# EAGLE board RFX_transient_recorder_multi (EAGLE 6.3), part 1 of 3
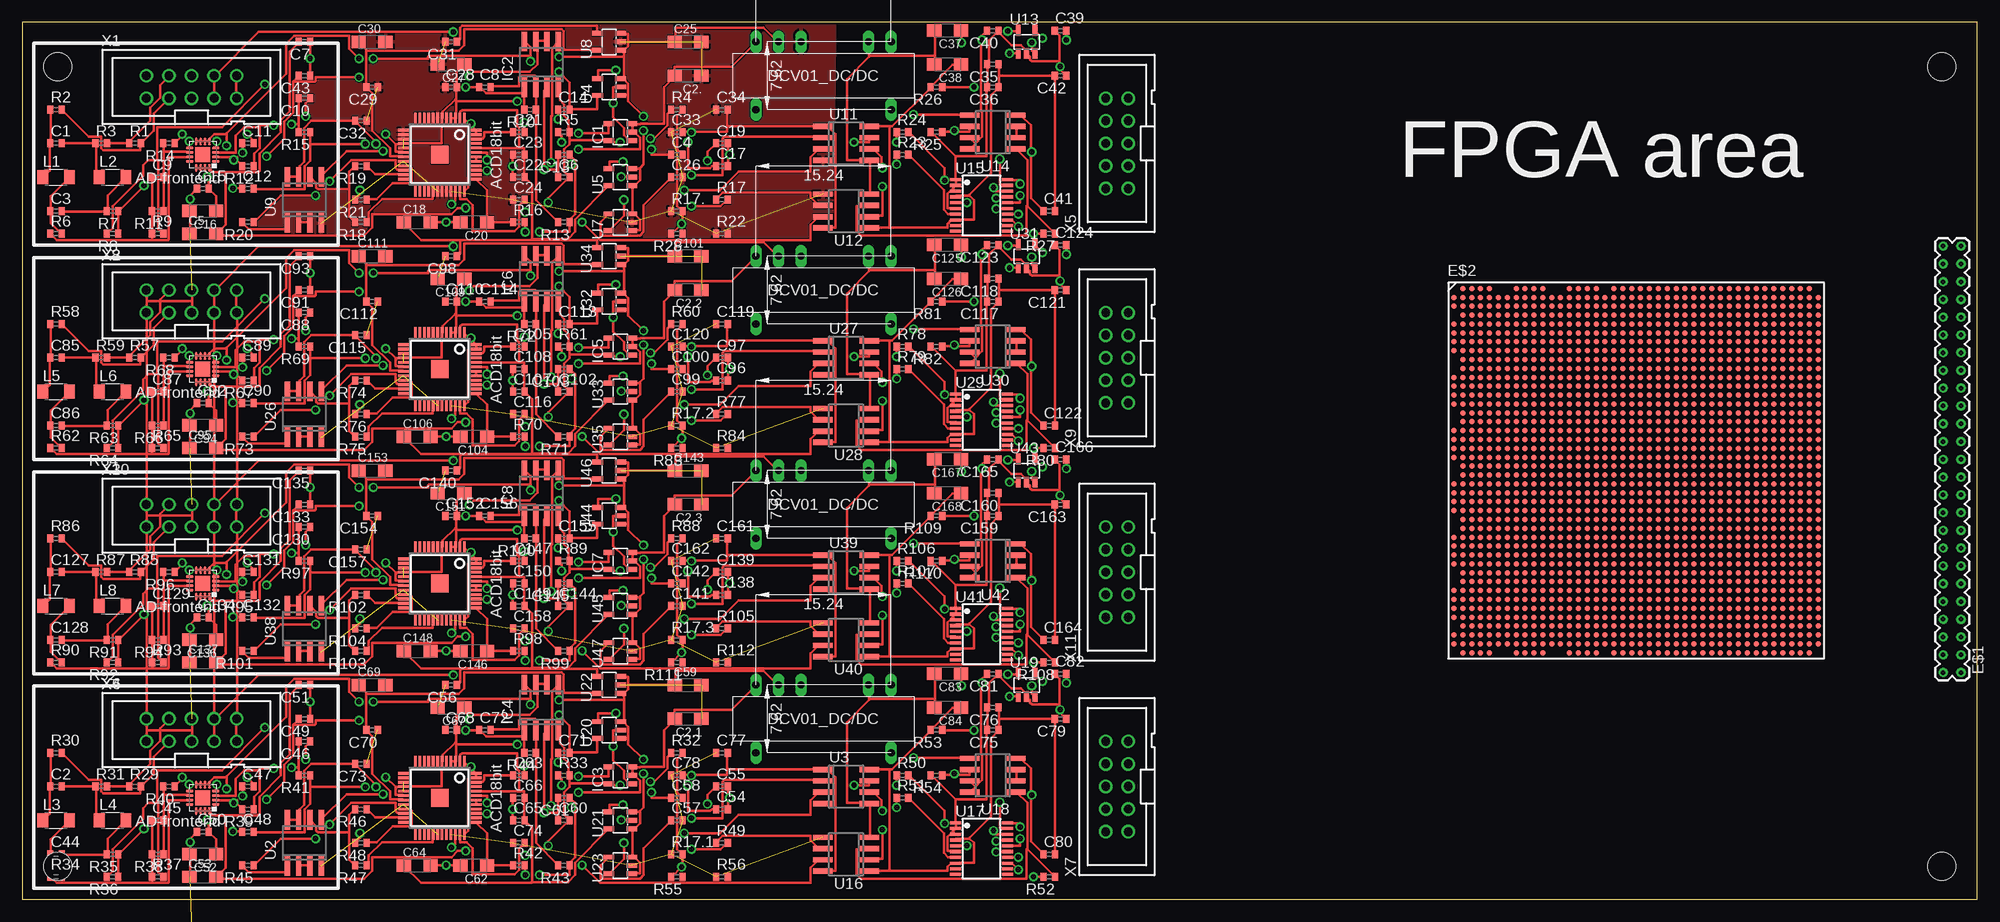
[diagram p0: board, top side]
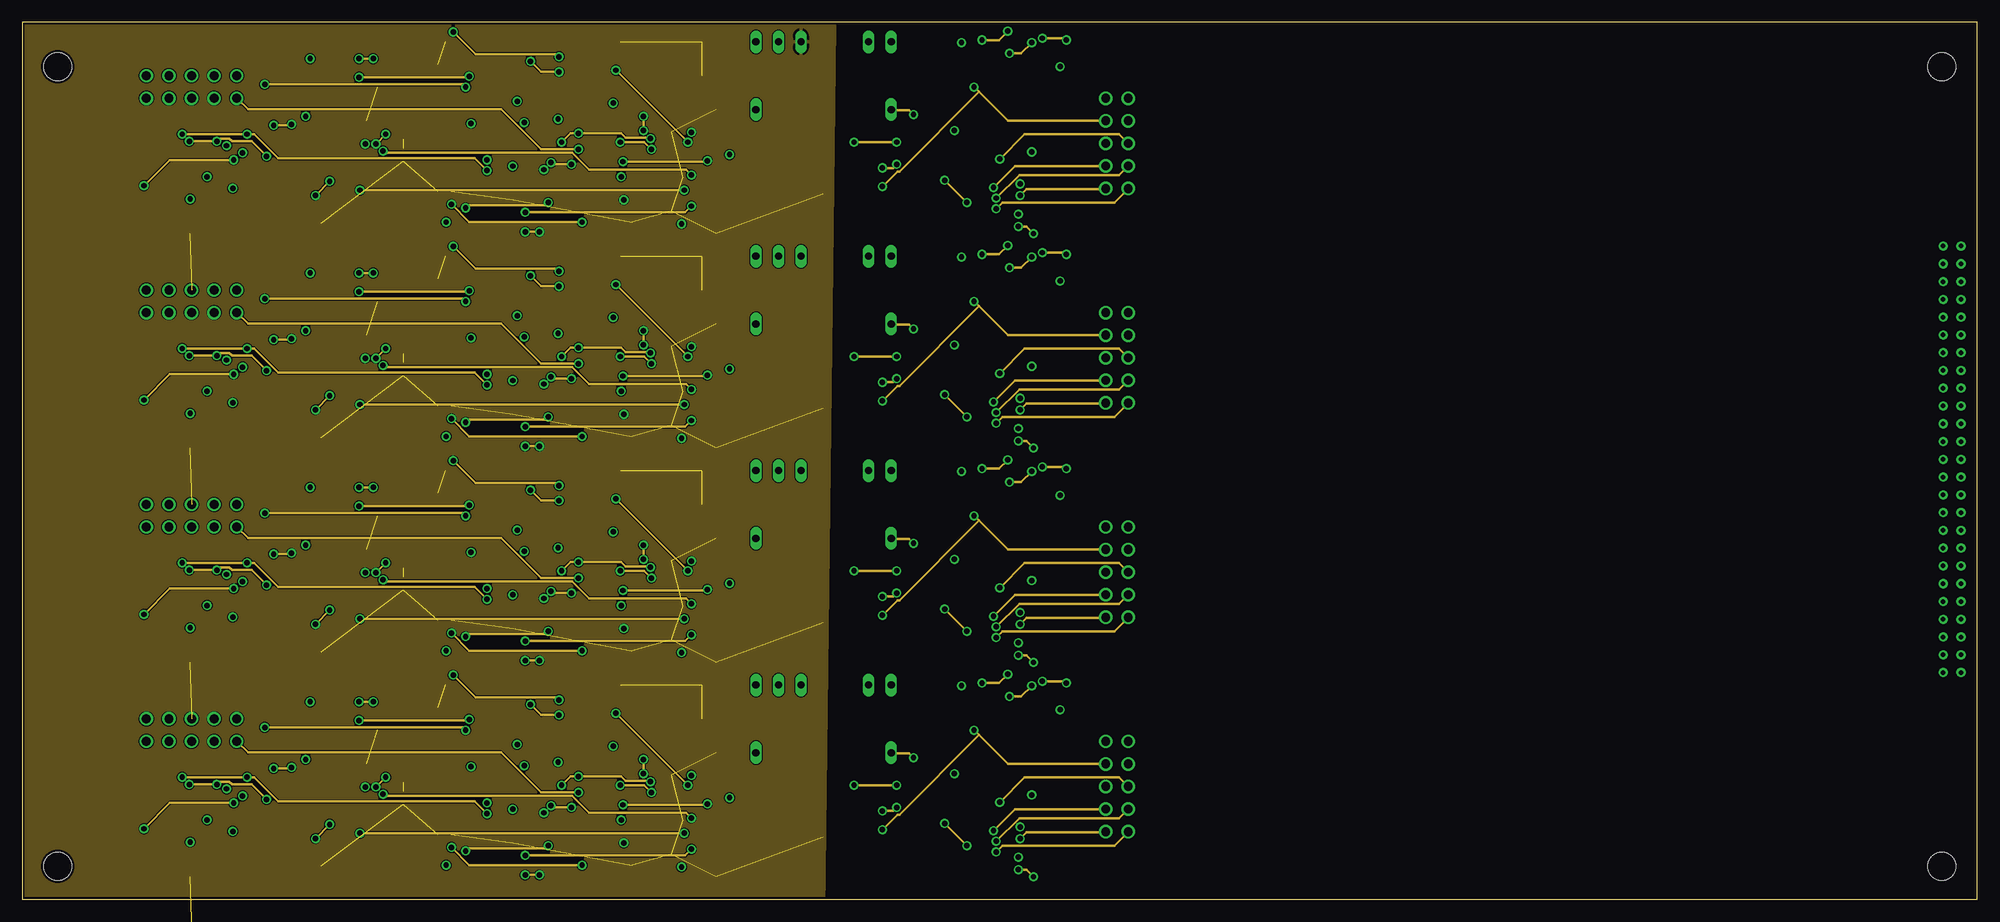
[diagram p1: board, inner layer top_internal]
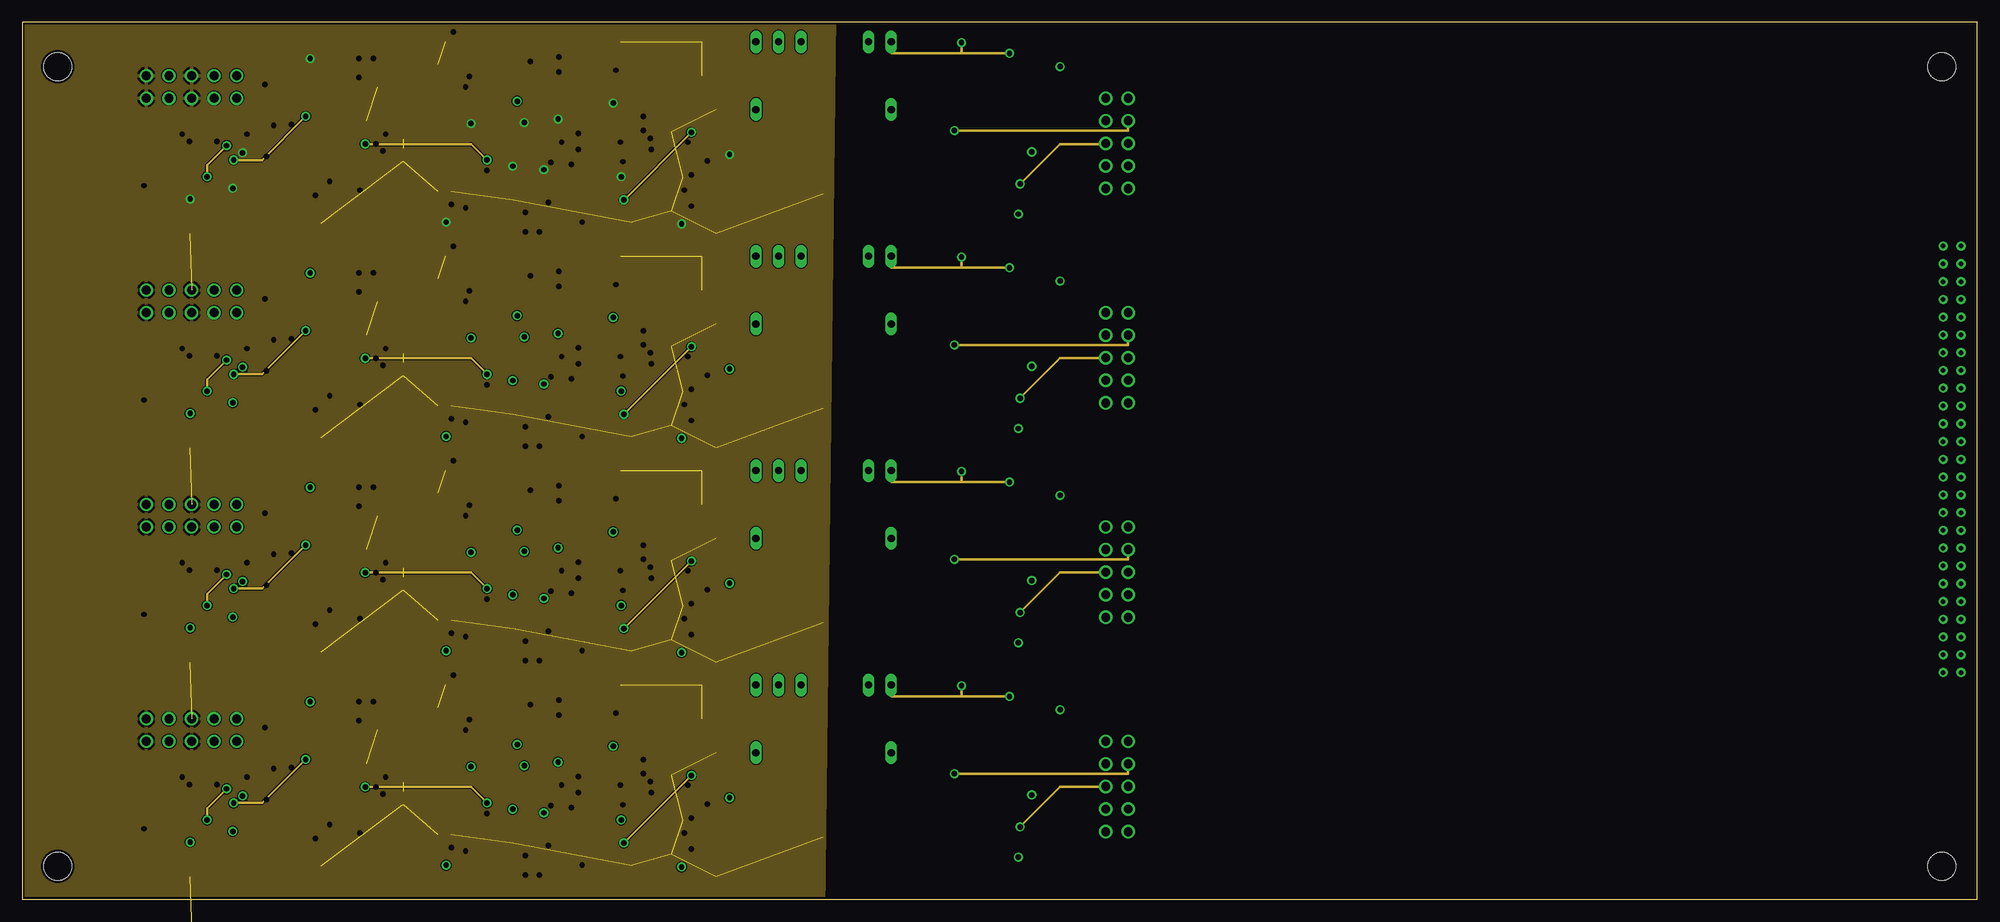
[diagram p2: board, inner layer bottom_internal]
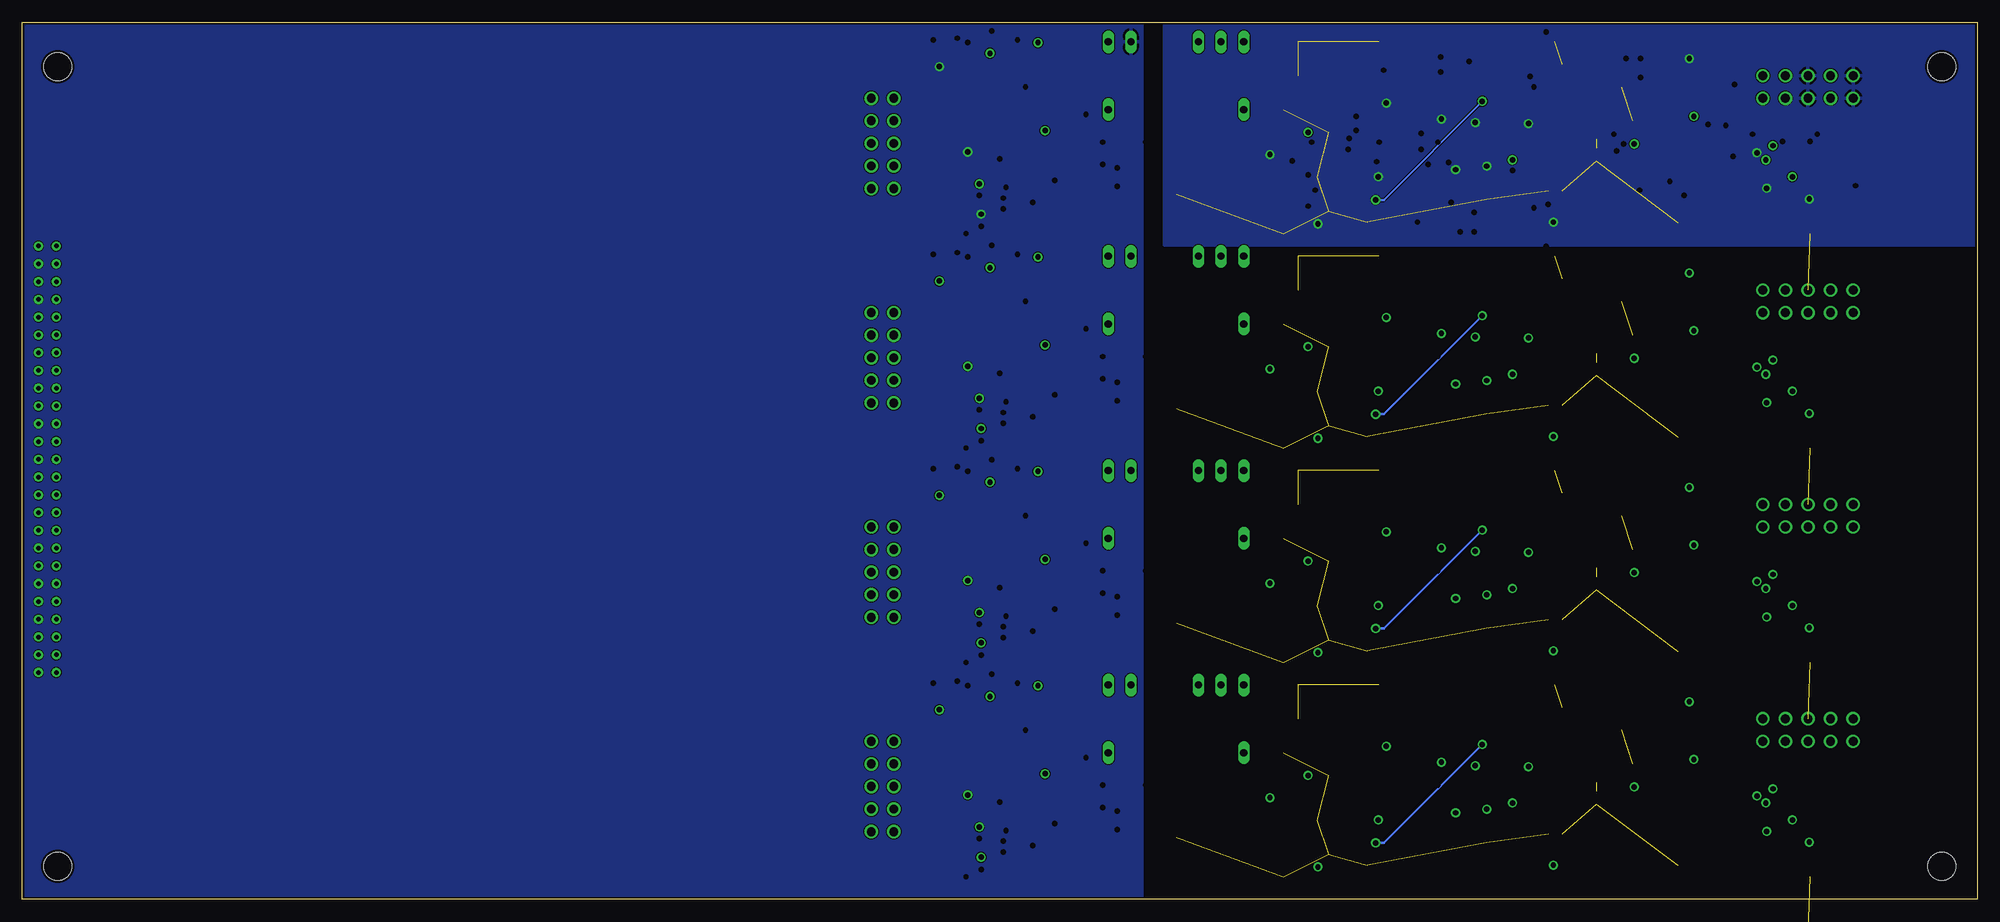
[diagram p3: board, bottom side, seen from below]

Size 220 x 98.73 mm. Coordinates in mm from the lower left corner, seen from the top.
Outline: 0,0 220,0 220,98.73 0,98.73 0,0
Copper layers ((1*2)+(15*16)): Top 0.035mm / dielectric 1.5mm / top_internal 0.035mm / dielectric 0.15mm / bottom_internal 0.035mm / dielectric 0.2mm / Bottom 0.035mm
Design rules "default *": minimum track width 10mil, minimum drill 24mil, track to track 4mil, track to pad 4mil, pad to pad 4mil, via to via 4mil, smd to smd 1mil, copper to edge 10mil, drill to drill 8mil, minimum pad ring 10mil, minimum via ring 8mil, stop-mask expansion 4mil, vias tented up to drill 0mil, thermal gap 10mil
Holes 3.2 mm at 4,93.73 4,3.73 216,93.73 216,3.73

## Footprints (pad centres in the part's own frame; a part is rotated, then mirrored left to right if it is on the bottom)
C0402 = smd 0.7 x 0.9: 1 -0.65,0; 2 0.65,0
SMC_A = smd 1.6 x 1.4: + -1.5,0; - 1.5,0
1297-25 = drill 0.508: A1 -24,-1; A2 -22,-1; A3 -20,-1; A4 -18,-1; A5 -16,-1; A6 -14,-1; A7 -12,-1; A8 -10,-1; A9 -8,-1; A10 -6,-1; A11 -4,-1; A12 -2,-1; A13 0,-1; A14 2,-1; A15 4,-1; A16 6,-1; A17 8,-1; A18 10,-1; A19 12,-1; A20 14,-1; A21 16,-1; A22 18,-1; A23 20,-1; A24 22,-1; A25 24,-1; B1 -24,1; B2 -22,1; B3 -20,1; B4 -18,1; B5 -16,1; B6 -14,1; B7 -12,1; B8 -10,1; B9 -8,1; B10 -6,1; B11 -4,1; B12 -2,1; B13 0,1; B14 2,1; B15 4,1; B16 6,1; B17 8,1; B18 10,1; B19 12,1; B20 14,1; B21 16,1; B22 18,1; B23 20,1; B24 22,1; B25 24,1
FF1738 = smd 0.6 x 0.6: A2 -19.5,20.5; A3 -18.5,20.5; A4 -17.5,20.5; A5 -16.5,20.5; A8 -13.5,20.5; A9 -12.5,20.5; A10 -11.5,20.5; A11 -10.5,20.5; A14 -7.5,20.5; A15 -6.5,20.5; A16 -5.5,20.5; A17 -4.5,20.5; A19 -2.5,20.5; A20 -1.5,20.5; A21 -0.5,20.5; A22 0.5,20.5; A23 1.5,20.5; A24 2.5,20.5; A25 3.5,20.5; A26 4.5,20.5; A27 5.5,20.5; A28 6.5,20.5; A29 7.5,20.5; A30 8.5,20.5; A31 9.5,20.5; A32 10.5,20.5; A33 11.5,20.5; A34 12.5,20.5; A35 13.5,20.5; A36 14.5,20.5; A37 15.5,20.5; A38 16.5,20.5; A39 17.5,20.5; A40 18.5,20.5; A41 19.5,20.5; AA2 -19.5,0.5; AA3 -18.5,0.5; AA4 -17.5,0.5; AA5 -16.5,0.5; AA6 -15.5,0.5; AA7 -14.5,0.5; AA8 -13.5,0.5; AA9 -12.5,0.5; AA10 -11.5,0.5; AA11 -10.5,0.5; AA12 -9.5,0.5; AA13 -8.5,0.5; AA14 -7.5,0.5; AA15 -6.5,0.5; AA16 -5.5,0.5; AA17 -4.5,0.5; AA18 -3.5,0.5; AA19 -2.5,0.5; AA20 -1.5,0.5; AA21 -0.5,0.5; AA22 0.5,0.5; AA23 1.5,0.5; AA24 2.5,0.5; AA25 3.5,0.5; AA26 4.5,0.5; AA27 5.5,0.5; AA28 6.5,0.5; AA29 7.5,0.5; AA30 8.5,0.5; AA31 9.5,0.5; AA32 10.5,0.5; AA33 11.5,0.5; AA34 12.5,0.5; AA35 13.5,0.5; AA36 14.5,0.5; AA37 15.5,0.5; AA38 16.5,0.5; AA39 17.5,0.5; AA40 18.5,0.5; AA41 19.5,0.5; AA42 20.5,0.5; AB2 -19.5,-0.5; AB3 -18.5,-0.5; AB4 -17.5,-0.5; AB5 -16.5,-0.5; AB6 -15.5,-0.5; AB7 -14.5,-0.5; AB8 -13.5,-0.5; AB9 -12.5,-0.5; AB10 -11.5,-0.5; AB11 -10.5,-0.5; AB12 -9.5,-0.5; AB13 -8.5,-0.5; AB14 -7.5,-0.5; AB15 -6.5,-0.5; AB16 -5.5,-0.5; AB17 -4.5,-0.5; AB18 -3.5,-0.5; AB19 -2.5,-0.5; AB20 -1.5,-0.5; AB21 -0.5,-0.5; AB22 0.5,-0.5; AB23 1.5,-0.5; AB24 2.5,-0.5; AB25 3.5,-0.5; AB26 4.5,-0.5; AB27 5.5,-0.5; AB28 6.5,-0.5; AB29 7.5,-0.5; AB30 8.5,-0.5; AB31 9.5,-0.5; AB32 10.5,-0.5; AB33 11.5,-0.5; AB34 12.5,-0.5; AB35 13.5,-0.5; AB36 14.5,-0.5; AB37 15.5,-0.5; AB38 16.5,-0.5; AB39 17.5,-0.5; AB40 18.5,-0.5; AB41 19.5,-0.5; AB42 20.5,-0.5; AC1 -20.5,-1.5; AC2 -19.5,-1.5; AC3 -18.5,-1.5; AC4 -17.5,-1.5; AC5 -16.5,-1.5; AC6 -15.5,-1.5; AC7 -14.5,-1.5; AC8 -13.5,-1.5; AC9 -12.5,-1.5; AC10 -11.5,-1.5; AC11 -10.5,-1.5; AC12 -9.5,-1.5; AC13 -8.5,-1.5; AC14 -7.5,-1.5; AC15 -6.5,-1.5; AC16 -5.5,-1.5; AC17 -4.5,-1.5; AC18 -3.5,-1.5; AC19 -2.5,-1.5; AC20 -1.5,-1.5; AC21 -0.5,-1.5; AC22 0.5,-1.5; AC23 1.5,-1.5; AC24 2.5,-1.5; AC25 3.5,-1.5; AC26 4.5,-1.5; AC27 5.5,-1.5; AC28 6.5,-1.5; AC29 7.5,-1.5; AC30 8.5,-1.5; AC31 9.5,-1.5; AC32 10.5,-1.5; AC33 11.5,-1.5; AC34 12.5,-1.5; AC35 13.5,-1.5; AC36 14.5,-1.5; AC37 15.5,-1.5; AC38 16.5,-1.5; AC39 17.5,-1.5; AC40 18.5,-1.5; AC41 19.5,-1.5; AC42 20.5,-1.5; AD1 -20.5,-2.5; AD2 -19.5,-2.5; AD3 -18.5,-2.5; AD4 -17.5,-2.5; AD5 -16.5,-2.5; AD6 -15.5,-2.5; AD7 -14.5,-2.5; AD8 -13.5,-2.5; AD9 -12.5,-2.5; AD10 -11.5,-2.5; AD11 -10.5,-2.5; AD12 -9.5,-2.5; AD13 -8.5,-2.5; AD14 -7.5,-2.5; AD15 -6.5,-2.5; AD16 -5.5,-2.5; AD17 -4.5,-2.5; AD18 -3.5,-2.5; AD19 -2.5,-2.5; AD20 -1.5,-2.5; AD21 -0.5,-2.5; AD22 0.5,-2.5; AD23 1.5,-2.5; AD24 2.5,-2.5; AD25 3.5,-2.5; AD26 4.5,-2.5; AD27 5.5,-2.5; AD28 6.5,-2.5; AD29 7.5,-2.5; AD30 8.5,-2.5; AD31 9.5,-2.5; AD32 10.5,-2.5; AD33 11.5,-2.5; AD34 12.5,-2.5; AD35 13.5,-2.5; AD36 14.5,-2.5; AD37 15.5,-2.5; AD38 16.5,-2.5; AD39 17.5,-2.5; AD40 18.5,-2.5; AD41 19.5,-2.5; AD42 20.5,-2.5; AE1 -20.5,-3.5; AE2 -19.5,-3.5; AE3 -18.5,-3.5; AE4 -17.5,-3.5; AE5 -16.5,-3.5; AE6 -15.5,-3.5; AE7 -14.5,-3.5; AE8 -13.5,-3.5; AE9 -12.5,-3.5; AE10 -11.5,-3.5; AE11 -10.5,-3.5; AE12 -9.5,-3.5; AE13 -8.5,-3.5; AE14 -7.5,-3.5; AE15 -6.5,-3.5; AE16 -5.5,-3.5; AE17 -4.5,-3.5; AE18 -3.5,-3.5; AE19 -2.5,-3.5; AE20 -1.5,-3.5; AE21 -0.5,-3.5; AE22 0.5,-3.5; AE23 1.5,-3.5; AE24 2.5,-3.5; AE25 3.5,-3.5; AE26 4.5,-3.5; AE27 5.5,-3.5; AE28 6.5,-3.5; AE29 7.5,-3.5; AE30 8.5,-3.5; AE31 9.5,-3.5; AE32 10.5,-3.5; AE33 11.5,-3.5; AE34 12.5,-3.5; AE35 13.5,-3.5; AE36 14.5,-3.5; AE37 15.5,-3.5; AE38 16.5,-3.5; AE39 17.5,-3.5; AE40 18.5,-3.5; AE41 19.5,-3.5; AE42 20.5,-3.5; AF1 -20.5,-4.5; AF2 -19.5,-4.5; AF3 -18.5,-4.5; AF4 -17.5,-4.5; AF5 -16.5,-4.5; AF6 -15.5,-4.5; AF7 -14.5,-4.5; AF8 -13.5,-4.5; AF9 -12.5,-4.5; AF10 -11.5,-4.5; AF11 -10.5,-4.5; AF12 -9.5,-4.5; AF13 -8.5,-4.5; AF14 -7.5,-4.5; AF15 -6.5,-4.5; AF16 -5.5,-4.5; AF17 -4.5,-4.5; AF18 -3.5,-4.5; AF19 -2.5,-4.5; AF20 -1.5,-4.5; AF21 -0.5,-4.5; AF22 0.5,-4.5; AF23 1.5,-4.5; AF24 2.5,-4.5; AF25 3.5,-4.5; AF26 4.5,-4.5; AF27 5.5,-4.5; AF28 6.5,-4.5; AF29 7.5,-4.5; AF30 8.5,-4.5; AF31 9.5,-4.5; AF32 10.5,-4.5; AF33 11.5,-4.5; AF34 12.5,-4.5; AF35 13.5,-4.5; AF36 14.5,-4.5; AF37 15.5,-4.5; AF38 16.5,-4.5; AF39 17.5,-4.5; AF40 18.5,-4.5; AF41 19.5,-4.5; AF42 20.5,-4.5; AG2 -19.5,-5.5; AG3 -18.5,-5.5; AG4 -17.5,-5.5; AG5 -16.5,-5.5; AG6 -15.5,-5.5; AG7 -14.5,-5.5; AG8 -13.5,-5.5; AG9 -12.5,-5.5; AG10 -11.5,-5.5; AG11 -10.5,-5.5; AG12 -9.5,-5.5; AG13 -8.5,-5.5; AG14 -7.5,-5.5; AG15 -6.5,-5.5; AG16 -5.5,-5.5; AG17 -4.5,-5.5; AG18 -3.5,-5.5; AG19 -2.5,-5.5; AG20 -1.5,-5.5; AG21 -0.5,-5.5; AG22 0.5,-5.5; AG23 1.5,-5.5; AG24 2.5,-5.5; AG25 3.5,-5.5; AG26 4.5,-5.5; AG27 5.5,-5.5; AG28 6.5,-5.5; AG29 7.5,-5.5; AG30 8.5,-5.5; AG31 9.5,-5.5; AG32 10.5,-5.5; AG33 11.5,-5.5; AG34 12.5,-5.5; AG35 13.5,-5.5; AG36 14.5,-5.5; AG37 15.5,-5.5; AG38 16.5,-5.5; AG39 17.5,-5.5; AG40 18.5,-5.5; AG41 19.5,-5.5; AG42 20.5,-5.5; AH2 -19.5,-6.5; AH3 -18.5,-6.5; AH4 -17.5,-6.5; AH5 -16.5,-6.5; AH6 -15.5,-6.5; AH7 -14.5,-6.5; AH8 -13.5,-6.5; AH9 -12.5,-6.5; AH10 -11.5,-6.5; AH11 -10.5,-6.5; AH12 -9.5,-6.5; AH13 -8.5,-6.5; AH14 -7.5,-6.5; AH15 -6.5,-6.5; AH16 -5.5,-6.5; AH17 -4.5,-6.5; AH18 -3.5,-6.5; AH19 -2.5,-6.5; AH20 -1.5,-6.5; AH21 -0.5,-6.5; AH22 0.5,-6.5; AH23 1.5,-6.5; AH24 2.5,-6.5; AH25 3.5,-6.5; AH26 4.5,-6.5; AH27 5.5,-6.5; AH28 6.5,-6.5; AH29 7.5,-6.5; AH30 8.5,-6.5; AH31 9.5,-6.5; AH32 10.5,-6.5; AH33 11.5,-6.5; AH34 12.5,-6.5; AH35 13.5,-6.5; AH36 14.5,-6.5; AH37 15.5,-6.5; AH38 16.5,-6.5; AH39 17.5,-6.5; AH40 18.5,-6.5; AH41 19.5,-6.5; AH42 20.5,-6.5; AJ1 -20.5,-7.5; AJ2 -19.5,-7.5; AJ3 -18.5,-7.5; AJ4 -17.5,-7.5; AJ5 -16.5,-7.5; AJ6 -15.5,-7.5; AJ7 -14.5,-7.5; AJ8 -13.5,-7.5; AJ9 -12.5,-7.5; AJ10 -11.5,-7.5; AJ11 -10.5,-7.5; AJ12 -9.5,-7.5; AJ13 -8.5,-7.5; AJ14 -7.5,-7.5; AJ15 -6.5,-7.5; AJ16 -5.5,-7.5; AJ17 -4.5,-7.5; AJ18 -3.5,-7.5; AJ19 -2.5,-7.5; AJ20 -1.5,-7.5; AJ21 -0.5,-7.5; AJ22 0.5,-7.5; AJ23 1.5,-7.5; AJ24 2.5,-7.5; AJ25 3.5,-7.5; AJ26 4.5,-7.5; AJ27 5.5,-7.5; AJ28 6.5,-7.5; AJ29 7.5,-7.5; AJ30 8.5,-7.5; AJ31 9.5,-7.5; AJ32 10.5,-7.5; AJ33 11.5,-7.5; AJ34 12.5,-7.5; AJ35 13.5,-7.5; AJ36 14.5,-7.5; AJ37 15.5,-7.5; AJ38 16.5,-7.5; AJ39 17.5,-7.5; AJ40 18.5,-7.5; AJ41 19.5,-7.5; AJ42 20.5,-7.5; AK1 -20.5,-8.5; AK2 -19.5,-8.5; AK3 -18.5,-8.5; AK4 -17.5,-8.5; AK5 -16.5,-8.5; AK6 -15.5,-8.5; AK7 -14.5,-8.5; AK8 -13.5,-8.5; AK9 -12.5,-8.5; AK10 -11.5,-8.5; AK11 -10.5,-8.5; AK12 -9.5,-8.5; AK13 -8.5,-8.5; AK14 -7.5,-8.5; AK15 -6.5,-8.5; AK16 -5.5,-8.5; AK17 -4.5,-8.5; AK18 -3.5,-8.5; AK19 -2.5,-8.5; AK20 -1.5,-8.5; AK21 -0.5,-8.5; AK22 0.5,-8.5; AK23 1.5,-8.5; AK24 2.5,-8.5; AK25 3.5,-8.5; AK26 4.5,-8.5; AK27 5.5,-8.5; AK28 6.5,-8.5; AK29 7.5,-8.5; AK30 8.5,-8.5; AK31 9.5,-8.5; AK32 10.5,-8.5; AK33 11.5,-8.5; AK34 12.5,-8.5; AK35 13.5,-8.5; AK36 14.5,-8.5; AK37 15.5,-8.5; AK38 16.5,-8.5; AK39 17.5,-8.5; AK40 18.5,-8.5; AK41 19.5,-8.5; AK42 20.5,-8.5; AL1 -20.5,-9.5; AL2 -19.5,-9.5; AL3 -18.5,-9.5; AL4 -17.5,-9.5; AL5 -16.5,-9.5; AL6 -15.5,-9.5; AL7 -14.5,-9.5; AL8 -13.5,-9.5; AL9 -12.5,-9.5; AL10 -11.5,-9.5; AL11 -10.5,-9.5; AL12 -9.5,-9.5; AL13 -8.5,-9.5; AL14 -7.5,-9.5; AL15 -6.5,-9.5; AL16 -5.5,-9.5; AL17 -4.5,-9.5; AL18 -3.5,-9.5; AL19 -2.5,-9.5; AL20 -1.5,-9.5; AL21 -0.5,-9.5; AL22 0.5,-9.5; AL23 1.5,-9.5; AL24 2.5,-9.5; AL25 3.5,-9.5; AL26 4.5,-9.5; AL27 5.5,-9.5; AL28 6.5,-9.5; AL29 7.5,-9.5; AL30 8.5,-9.5; AL31 9.5,-9.5; AL32 10.5,-9.5; AL33 11.5,-9.5; AL34 12.5,-9.5; AL35 13.5,-9.5; AL36 14.5,-9.5; AL37 15.5,-9.5; AL38 16.5,-9.5; AL39 17.5,-9.5; AL40 18.5,-9.5; AL41 19.5,-9.5; AL42 20.5,-9.5; AM1 -20.5,-10.5; AM2 -19.5,-10.5; AM3 -18.5,-10.5; AM4 -17.5,-10.5; AM5 -16.5,-10.5; AM6 -15.5,-10.5; AM7 -14.5,-10.5; AM8 -13.5,-10.5; AM9 -12.5,-10.5; AM10 -11.5,-10.5; AM11 -10.5,-10.5; AM12 -9.5,-10.5; AM13 -8.5,-10.5; AM14 -7.5,-10.5; AM15 -6.5,-10.5; AM16 -5.5,-10.5; AM17 -4.5,-10.5; AM18 -3.5,-10.5; AM19 -2.5,-10.5; AM20 -1.5,-10.5; AM21 -0.5,-10.5; AM22 0.5,-10.5; AM23 1.5,-10.5; AM24 2.5,-10.5; AM25 3.5,-10.5; AM26 4.5,-10.5; AM27 5.5,-10.5; AM28 6.5,-10.5; AM29 7.5,-10.5; AM30 8.5,-10.5; AM31 9.5,-10.5; AM32 10.5,-10.5; AM33 11.5,-10.5; AM34 12.5,-10.5; AM35 13.5,-10.5; AM36 14.5,-10.5; AM37 15.5,-10.5; AM38 16.5,-10.5; AM39 17.5,-10.5; AM40 18.5,-10.5; AM41 19.5,-10.5; AM42 20.5,-10.5; AN2 -19.5,-11.5; AN3 -18.5,-11.5; AN4 -17.5,-11.5; AN5 -16.5,-11.5; AN6 -15.5,-11.5; AN7 -14.5,-11.5; AN8 -13.5,-11.5; AN9 -12.5,-11.5; AN10 -11.5,-11.5; AN11 -10.5,-11.5; AN12 -9.5,-11.5; AN13 -8.5,-11.5; AN14 -7.5,-11.5; AN15 -6.5,-11.5; AN16 -5.5,-11.5; AN17 -4.5,-11.5; AN18 -3.5,-11.5; AN19 -2.5,-11.5; AN20 -1.5,-11.5; AN21 -0.5,-11.5; AN22 0.5,-11.5; AN23 1.5,-11.5; AN24 2.5,-11.5; AN25 3.5,-11.5; AN26 4.5,-11.5; AN27 5.5,-11.5; AN28 6.5,-11.5; AN29 7.5,-11.5; AN30 8.5,-11.5; AN31 9.5,-11.5; AN32 10.5,-11.5; AN33 11.5,-11.5; AN34 12.5,-11.5; AN35 13.5,-11.5; AN36 14.5,-11.5; AN37 15.5,-11.5; AN38 16.5,-11.5; AN39 17.5,-11.5; AN40 18.5,-11.5; AN41 19.5,-11.5; AN42 20.5,-11.5; AP2 -19.5,-12.5; AP3 -18.5,-12.5; AP4 -17.5,-12.5; AP5 -16.5,-12.5; AP6 -15.5,-12.5; AP7 -14.5,-12.5; AP8 -13.5,-12.5; AP9 -12.5,-12.5; AP10 -11.5,-12.5; AP11 -10.5,-12.5; AP12 -9.5,-12.5; AP13 -8.5,-12.5; AP14 -7.5,-12.5; AP15 -6.5,-12.5; AP16 -5.5,-12.5; AP17 -4.5,-12.5; AP18 -3.5,-12.5; AP19 -2.5,-12.5; AP20 -1.5,-12.5; AP21 -0.5,-12.5; AP22 0.5,-12.5; AP23 1.5,-12.5; AP24 2.5,-12.5; AP25 3.5,-12.5; AP26 4.5,-12.5; AP27 5.5,-12.5; AP28 6.5,-12.5; AP29 7.5,-12.5; AP30 8.5,-12.5; AP31 9.5,-12.5; AP32 10.5,-12.5; AP33 11.5,-12.5; AP34 12.5,-12.5; AP35 13.5,-12.5; AP36 14.5,-12.5; AP37 15.5,-12.5; AP38 16.5,-12.5; AP39 17.5,-12.5; AP40 18.5,-12.5; AP41 19.5,-12.5; AP42 20.5,-12.5; AR1 -20.5,-13.5; AR2 -19.5,-13.5; AR3 -18.5,-13.5; AR4 -17.5,-13.5; AR5 -16.5,-13.5; AR6 -15.5,-13.5; AR7 -14.5,-13.5; AR8 -13.5,-13.5; AR9 -12.5,-13.5; AR10 -11.5,-13.5; AR11 -10.5,-13.5; AR12 -9.5,-13.5; AR13 -8.5,-13.5; AR14 -7.5,-13.5; AR15 -6.5,-13.5; AR16 -5.5,-13.5; AR17 -4.5,-13.5; AR18 -3.5,-13.5; AR19 -2.5,-13.5; AR20 -1.5,-13.5; AR21 -0.5,-13.5; AR22 0.5,-13.5; AR23 1.5,-13.5; AR24 2.5,-13.5; AR25 3.5,-13.5; AR26 4.5,-13.5; AR27 5.5,-13.5; AR28 6.5,-13.5; AR29 7.5,-13.5; AR30 8.5,-13.5; AR31 9.5,-13.5; AR32 10.5,-13.5; AR33 11.5,-13.5; AR34 12.5,-13.5; AR35 13.5,-13.5; AR36 14.5,-13.5; AR37 15.5,-13.5; AR38 16.5,-13.5; AR39 17.5,-13.5; AR40 18.5,-13.5; AR41 19.5,-13.5; AR42 20.5,-13.5; AT1 -20.5,-14.5; AT2 -19.5,-14.5; AT3 -18.5,-14.5; AT4 -17.5,-14.5; AT5 -16.5,-14.5; AT6 -15.5,-14.5; AT7 -14.5,-14.5; AT8 -13.5,-14.5; AT9 -12.5,-14.5; AT10 -11.5,-14.5; AT11 -10.5,-14.5; AT12 -9.5,-14.5; AT13 -8.5,-14.5; AT14 -7.5,-14.5; AT15 -6.5,-14.5; AT16 -5.5,-14.5; AT17 -4.5,-14.5; AT18 -3.5,-14.5; AT19 -2.5,-14.5; AT20 -1.5,-14.5; AT21 -0.5,-14.5; AT22 0.5,-14.5; AT23 1.5,-14.5; AT24 2.5,-14.5; AT25 3.5,-14.5; AT26 4.5,-14.5; AT27 5.5,-14.5; AT28 6.5,-14.5; AT29 7.5,-14.5; AT30 8.5,-14.5; AT31 9.5,-14.5; AT32 10.5,-14.5; AT33 11.5,-14.5; AT34 12.5,-14.5; AT35 13.5,-14.5; AT36 14.5,-14.5; AT37 15.5,-14.5; AT38 16.5,-14.5; AT39 17.5,-14.5; AT40 18.5,-14.5; AT41 19.5,-14.5; AT42 20.5,-14.5; AU1 -20.5,-15.5; AU2 -19.5,-15.5; AU3 -18.5,-15.5; AU4 -17.5,-15.5; AU5 -16.5,-15.5; AU6 -15.5,-15.5; AU7 -14.5,-15.5; AU8 -13.5,-15.5; AU9 -12.5,-15.5; AU10 -11.5,-15.5; AU11 -10.5,-15.5; AU12 -9.5,-15.5; AU13 -8.5,-15.5; AU14 -7.5,-15.5; AU15 -6.5,-15.5; AU16 -5.5,-15.5; AU17 -4.5,-15.5; AU18 -3.5,-15.5; AU19 -2.5,-15.5; AU20 -1.5,-15.5; AU21 -0.5,-15.5; AU22 0.5,-15.5; AU23 1.5,-15.5; AU24 2.5,-15.5; AU25 3.5,-15.5; AU26 4.5,-15.5; AU27 5.5,-15.5; AU28 6.5,-15.5; AU29 7.5,-15.5; AU30 8.5,-15.5; AU31 9.5,-15.5; AU32 10.5,-15.5; AU33 11.5,-15.5; AU34 12.5,-15.5; AU35 13.5,-15.5; AU36 14.5,-15.5; AU37 15.5,-15.5; AU38 16.5,-15.5; AU39 17.5,-15.5; AU40 18.5,-15.5; AU41 19.5,-15.5; AU42 20.5,-15.5; AV1 -20.5,-16.5; AV2 -19.5,-16.5; AV3 -18.5,-16.5; AV4 -17.5,-16.5; AV5 -16.5,-16.5; AV6 -15.5,-16.5; AV7 -14.5,-16.5; AV8 -13.5,-16.5; AV9 -12.5,-16.5; AV10 -11.5,-16.5; AV11 -10.5,-16.5; AV12 -9.5,-16.5; AV13 -8.5,-16.5; AV14 -7.5,-16.5; AV15 -6.5,-16.5; AV16 -5.5,-16.5; AV17 -4.5,-16.5; AV18 -3.5,-16.5; AV19 -2.5,-16.5; AV20 -1.5,-16.5; AV21 -0.5,-16.5; AV22 0.5,-16.5; AV23 1.5,-16.5; AV24 2.5,-16.5; AV25 3.5,-16.5; AV26 4.5,-16.5; AV27 5.5,-16.5; AV28 6.5,-16.5; AV29 7.5,-16.5; AV30 8.5,-16.5; AV31 9.5,-16.5; AV32 10.5,-16.5; AV33 11.5,-16.5; AV34 12.5,-16.5; AV35 13.5,-16.5; AV36 14.5,-16.5; AV37 15.5,-16.5; AV38 16.5,-16.5; AV39 17.5,-16.5; AV40 18.5,-16.5; AV41 19.5,-16.5; AV42 20.5,-16.5; AW2 -19.5,-17.5; AW3 -18.5,-17.5; AW4 -17.5,-17.5; AW5 -16.5,-17.5; AW6 -15.5,-17.5; AW7 -14.5,-17.5; AW8 -13.5,-17.5; AW9 -12.5,-17.5; AW10 -11.5,-17.5; AW11 -10.5,-17.5; AW12 -9.5,-17.5; AW13 -8.5,-17.5; AW14 -7.5,-17.5; AW15 -6.5,-17.5; AW16 -5.5,-17.5; AW17 -4.5,-17.5; AW18 -3.5,-17.5; AW19 -2.5,-17.5; AW20 -1.5,-17.5; AW21 -0.5,-17.5; AW22 0.5,-17.5; AW23 1.5,-17.5; AW24 2.5,-17.5; AW25 3.5,-17.5; AW26 4.5,-17.5; AW27 5.5,-17.5; AW28 6.5,-17.5; AW29 7.5,-17.5; AW30 8.5,-17.5; AW31 9.5,-17.5; AW32 10.5,-17.5; AW33 11.5,-17.5; AW34 12.5,-17.5; AW35 13.5,-17.5; AW36 14.5,-17.5; AW37 15.5,-17.5; AW38 16.5,-17.5; AW39 17.5,-17.5; AW40 18.5,-17.5; AW41 19.5,-17.5; AW42 20.5,-17.5; AY1 -20.5,-18.5; AY2 -19.5,-18.5; AY3 -18.5,-18.5; AY4 -17.5,-18.5; AY5 -16.5,-18.5; AY6 -15.5,-18.5; AY7 -14.5,-18.5; AY8 -13.5,-18.5; AY9 -12.5,-18.5; AY10 -11.5,-18.5; AY11 -10.5,-18.5; AY12 -9.5,-18.5; AY13 -8.5,-18.5; AY14 -7.5,-18.5; AY15 -6.5,-18.5; AY16 -5.5,-18.5; AY17 -4.5,-18.5; AY18 -3.5,-18.5; AY19 -2.5,-18.5; AY20 -1.5,-18.5; AY21 -0.5,-18.5; AY22 0.5,-18.5; AY23 1.5,-18.5; AY24 2.5,-18.5; AY25 3.5,-18.5; AY26 4.5,-18.5; AY27 5.5,-18.5; AY28 6.5,-18.5; AY29 7.5,-18.5; AY30 8.5,-18.5; AY31 9.5,-18.5; AY32 10.5,-18.5; AY33 11.5,-18.5; AY34 12.5,-18.5; AY35 13.5,-18.5; AY36 14.5,-18.5; AY37 15.5,-18.5; AY38 16.5,-18.5; AY39 17.5,-18.5; AY40 18.5,-18.5; AY41 19.5,-18.5; AY42 20.5,-18.5; B1 -20.5,19.5; B2 -19.5,19.5; B3 -18.5,19.5; B4 -17.5,19.5; B5 -16.5,19.5; B6 -15.5,19.5; B7 -14.5,19.5; B8 -13.5,19.5; B9 -12.5,19.5; B10 -11.5,19.5; B11 -10.5,19.5; B12 -9.5,19.5; B13 -8.5,19.5; B14 -7.5,19.5; B15 -6.5,19.5; B16 -5.5,19.5; B17 -4.5,19.5; B18 -3.5,19.5; B19 -2.5,19.5; B20 -1.5,19.5; B21 -0.5,19.5; B22 0.5,19.5; B23 1.5,19.5; B24 2.5,19.5; B25 3.5,19.5; B26 4.5,19.5; B27 5.5,19.5; B28 6.5,19.5; B29 7.5,19.5; B30 8.5,19.5; B31 9.5,19.5; B32 10.5,19.5; B33 11.5,19.5; B34 12.5,19.5; B35 13.5,19.5; B36 14.5,19.5; B37 15.5,19.5; B38 16.5,19.5; B39 17.5,19.5; B40 18.5,19.5; B41 19.5,19.5; B42 20.5,19.5; BA1 -20.5,-19.5; BA2 -19.5,-19.5; BA3 -18.5,-19.5; BA4 -17.5,-19.5; BA5 -16.5,-19.5; BA6 -15.5,-19.5; BA7 -14.5,-19.5; BA8 -13.5,-19.5; BA9 -12.5,-19.5; BA10 -11.5,-19.5; BA11 -10.5,-19.5; BA12 -9.5,-19.5; BA13 -8.5,-19.5; BA14 -7.5,-19.5; BA15 -6.5,-19.5; BA16 -5.5,-19.5; BA17 -4.5,-19.5; BA18 -3.5,-19.5; BA19 -2.5,-19.5; BA20 -1.5,-19.5; BA21 -0.5,-19.5; BA22 0.5,-19.5; BA23 1.5,-19.5; BA24 2.5,-19.5; BA25 3.5,-19.5; BA26 4.5,-19.5; BA27 5.5,-19.5; BA28 6.5,-19.5; BA29 7.5,-19.5; BA30 8.5,-19.5; BA31 9.5,-19.5; BA32 10.5,-19.5; BA33 11.5,-19.5; BA34 12.5,-19.5; BA35 13.5,-19.5; BA36 14.5,-19.5; BA37 15.5,-19.5; BA38 16.5,-19.5; BA39 17.5,-19.5; BA40 18.5,-19.5; BA41 19.5,-19.5; BA42 20.5,-19.5; BB2 -19.5,-20.5; BB3 -18.5,-20.5; BB4 -17.5,-20.5; BB5 -16.5,-20.5; BB8 -13.5,-20.5; BB9 -12.5,-20.5; BB10 -11.5,-20.5; BB11 -10.5,-20.5; BB14 -7.5,-20.5; BB15 -6.5,-20.5; BB16 -5.5,-20.5; BB17 -4.5,-20.5; BB19 -2.5,-20.5; BB20 -1.5,-20.5; BB21 -0.5,-20.5; BB22 0.5,-20.5; BB23 1.5,-20.5; BB24 2.5,-20.5; BB25 3.5,-20.5; BB26 4.5,-20.5; BB27 5.5,-20.5; BB28 6.5,-20.5; BB29 7.5,-20.5; BB30 8.5,-20.5; BB31 9.5,-20.5; BB32 10.5,-20.5; BB33 11.5,-20.5; BB34 12.5,-20.5; BB35 13.5,-20.5; BB36 14.5,-20.5; BB37 15.5,-20.5; BB38 16.5,-20.5; BB39 17.5,-20.5; BB40 18.5,-20.5; BB41 19.5,-20.5; C1 -20.5,18.5; C2 -19.5,18.5; C3 -18.5,18.5; C4 -17.5,18.5; C5 -16.5,18.5; C6 -15.5,18.5; C7 -14.5,18.5; C8 -13.5,18.5; C9 -12.5,18.5; C10 -11.5,18.5; C11 -10.5,18.5; C12 -9.5,18.5; C13 -8.5,18.5; C14 -7.5,18.5; C15 -6.5,18.5; C16 -5.5,18.5; C17 -4.5,18.5; C18 -3.5,18.5; C19 -2.5,18.5; C20 -1.5,18.5; C21 -0.5,18.5; C22 0.5,18.5; C23 1.5,18.5; C24 2.5,18.5; C25 3.5,18.5; C26 4.5,18.5; C27 5.5,18.5; C28 6.5,18.5; C29 7.5,18.5; C30 8.5,18.5; C31 9.5,18.5; C32 10.5,18.5; C33 11.5,18.5; C34 12.5,18.5; C35 13.5,18.5; C36 14.5,18.5; C37 15.5,18.5; C38 16.5,18.5; C39 17.5,18.5; C40 18.5,18.5; C41 19.5,18.5; C42 20.5,18.5; D2 -19.5,17.5; D3 -18.5,17.5; D4 -17.5,17.5; D5 -16.5,17.5; D6 -15.5,17.5; D7 -14.5,17.5; D8 -13.5,17.5; D9 -12.5,17.5; D10 -11.5,17.5; D11 -10.5,17.5; D12 -9.5,17.5; D13 -8.5,17.5; D14 -7.5,17.5; D15 -6.5,17.5; D16 -5.5,17.5; D17 -4.5,17.5; D18 -3.5,17.5; D19 -2.5,17.5; D20 -1.5,17.5; D21 -0.5,17.5; D22 0.5,17.5; D23 1.5,17.5; D24 2.5,17.5; D25 3.5,17.5; D26 4.5,17.5; D27 5.5,17.5; D28 6.5,17.5; D29 7.5,17.5; D30 8.5,17.5; D31 9.5,17.5; D32 10.5,17.5; D33 11.5,17.5; D34 12.5,17.5; D35 13.5,17.5; D36 14.5,17.5; D37 15.5,17.5; D38 16.5,17.5; D39 17.5,17.5; D40 18.5,17.5; D41 19.5,17.5; D42 20.5,17.5; E1 -20.5,16.5; E2 -19.5,16.5; E3 -18.5,16.5; E4 -17.5,16.5; E5 -16.5,16.5; E6 -15.5,16.5; E7 -14.5,16.5; E8 -13.5,16.5; E9 -12.5,16.5; E10 -11.5,16.5; E11 -10.5,16.5; E12 -9.5,16.5; E13 -8.5,16.5; E14 -7.5,16.5; E15 -6.5,16.5; E16 -5.5,16.5; E17 -4.5,16.5; E18 -3.5,16.5; E19 -2.5,16.5; E20 -1.5,16.5; E21 -0.5,16.5; E22 0.5,16.5; E23 1.5,16.5; E24 2.5,16.5; E25 3.5,16.5; E26 4.5,16.5; E27 5.5,16.5; E28 6.5,16.5; E29 7.5,16.5; E30 8.5,16.5; E31 9.5,16.5; E32 10.5,16.5; E33 11.5,16.5; E34 12.5,16.5; E35 13.5,16.5; E36 14.5,16.5; E37 15.5,16.5; E38 16.5,16.5; E39 17.5,16.5; E40 18.5,16.5; E41 19.5,16.5; E42 20.5,16.5; F1 -20.5,15.5; F2 -19.5,15.5; F3 -18.5,15.5; F4 -17.5,15.5; F5 -16.5,15.5; F6 -15.5,15.5; F7 -14.5,15.5; F8 -13.5,15.5; F9 -12.5,15.5; F10 -11.5,15.5; F11 -10.5,15.5; F12 -9.5,15.5; F13 -8.5,15.5; F14 -7.5,15.5; F15 -6.5,15.5; F16 -5.5,15.5; F17 -4.5,15.5; F18 -3.5,15.5; F19 -2.5,15.5; F20 -1.5,15.5; F21 -0.5,15.5; F22 0.5,15.5; F23 1.5,15.5; F24 2.5,15.5; F25 3.5,15.5; F26 4.5,15.5; F27 5.5,15.5; F28 6.5,15.5; F29 7.5,15.5; F30 8.5,15.5; F31 9.5,15.5; F32 10.5,15.5; F33 11.5,15.5; F34 12.5,15.5; F35 13.5,15.5; F36 14.5,15.5; F37 15.5,15.5; F38 16.5,15.5; F39 17.5,15.5; F40 18.5,15.5; F41 19.5,15.5; F42 20.5,15.5; G1 -20.5,14.5; G2 -19.5,14.5; G3 -18.5,14.5; G4 -17.5,14.5; G5 -16.5,14.5; G6 -15.5,14.5; G7 -14.5,14.5; G8 -13.5,14.5; G9 -12.5,14.5; G10 -11.5,14.5; G11 -10.5,14.5; G12 -9.5,14.5; G13 -8.5,14.5; G14 -7.5,14.5; G15 -6.5,14.5; G16 -5.5,14.5; G17 -4.5,14.5; G18 -3.5,14.5; G19 -2.5,14.5; G20 -1.5,14.5; G21 -0.5,14.5; G22 0.5,14.5; G23 1.5,14.5; G24 2.5,14.5; G25 3.5,14.5; G26 4.5,14.5; G27 5.5,14.5; G28 6.5,14.5; G29 7.5,14.5; G30 8.5,14.5; G31 9.5,14.5; G32 10.5,14.5; G33 11.5,14.5; G34 12.5,14.5; G35 13.5,14.5; G36 14.5,14.5; G37 15.5,14.5; G38 16.5,14.5; G39 17.5,14.5; G40 18.5,14.5; G41 19.5,14.5; G42 20.5,14.5; H1 -20.5,13.5; H2 -19.5,13.5; H3 -18.5,13.5; H4 -17.5,13.5; H5 -16.5,13.5; H6 -15.5,13.5; H7 -14.5,13.5; H8 -13.5,13.5; H9 -12.5,13.5; H10 -11.5,13.5; H11 -10.5,13.5; H12 -9.5,13.5; H13 -8.5,13.5; H14 -7.5,13.5; H15 -6.5,13.5; H16 -5.5,13.5; H17 -4.5,13.5; H18 -3.5,13.5; H19 -2.5,13.5; H20 -1.5,13.5; H21 -0.5,13.5; H22 0.5,13.5; H23 1.5,13.5; H24 2.5,13.5; H25 3.5,13.5; H26 4.5,13.5; H27 5.5,13.5; H28 6.5,13.5; H29 7.5,13.5; H30 8.5,13.5; H31 9.5,13.5; H32 10.5,13.5; H33 11.5,13.5; H34 12.5,13.5; H35 13.5,13.5; H36 14.5,13.5; H37 15.5,13.5; H38 16.5,13.5; H39 17.5,13.5; H40 18.5,13.5; H41 19.5,13.5; H42 20.5,13.5; J2 -19.5,12.5; J3 -18.5,12.5; J4 -17.5,12.5; J5 -16.5,12.5; J6 -15.5,12.5; J7 -14.5,12.5; J8 -13.5,12.5; J9 -12.5,12.5; J10 -11.5,12.5; J11 -10.5,12.5; J12 -9.5,12.5; J13 -8.5,12.5; J14 -7.5,12.5; J15 -6.5,12.5; J16 -5.5,12.5; J17 -4.5,12.5; J18 -3.5,12.5; J19 -2.5,12.5; J20 -1.5,12.5; J21 -0.5,12.5; J22 0.5,12.5; J23 1.5,12.5; J24 2.5,12.5; J25 3.5,12.5; J26 4.5,12.5; J27 5.5,12.5; J28 6.5,12.5; J29 7.5,12.5; J30 8.5,12.5; J31 9.5,12.5; J32 10.5,12.5; J33 11.5,12.5; J34 12.5,12.5; J35 13.5,12.5; J36 14.5,12.5; J37 15.5,12.5; J38 16.5,12.5; J39 17.5,12.5; J40 18.5,12.5; J41 19.5,12.5; J42 20.5,12.5; K2 -19.5,11.5; K3 -18.5,11.5; K4 -17.5,11.5; K5 -16.5,11.5; K6 -15.5,11.5; K7 -14.5,11.5; K8 -13.5,11.5; K9 -12.5,11.5; K10 -11.5,11.5; K11 -10.5,11.5; K12 -9.5,11.5; K13 -8.5,11.5; K14 -7.5,11.5; K15 -6.5,11.5; K16 -5.5,11.5; K17 -4.5,11.5; K18 -3.5,11.5; K19 -2.5,11.5; K20 -1.5,11.5; K21 -0.5,11.5; K22 0.5,11.5; K23 1.5,11.5; K24 2.5,11.5; K25 3.5,11.5; K26 4.5,11.5; K27 5.5,11.5; K28 6.5,11.5; K29 7.5,11.5; K30 8.5,11.5; K31 9.5,11.5; K32 10.5,11.5; K33 11.5,11.5; K34 12.5,11.5; K35 13.5,11.5; K36 14.5,11.5; K37 15.5,11.5; K38 16.5,11.5; K39 17.5,11.5; K40 18.5,11.5; K41 19.5,11.5; K42 20.5,11.5; L1 -20.5,10.5; L2 -19.5,10.5; L3 -18.5,10.5; L4 -17.5,10.5; L5 -16.5,10.5; L6 -15.5,10.5; L7 -14.5,10.5; L8 -13.5,10.5; L9 -12.5,10.5; L10 -11.5,10.5; L11 -10.5,10.5; L12 -9.5,10.5; L13 -8.5,10.5; L14 -7.5,10.5; L15 -6.5,10.5; L16 -5.5,10.5; L17 -4.5,10.5; L18 -3.5,10.5; L19 -2.5,10.5; L20 -1.5,10.5; L21 -0.5,10.5; L22 0.5,10.5; L23 1.5,10.5; L24 2.5,10.5; L25 3.5,10.5; L26 4.5,10.5; L27 5.5,10.5; L28 6.5,10.5; L29 7.5,10.5; L30 8.5,10.5; L31 9.5,10.5; L32 10.5,10.5; L33 11.5,10.5; L34 12.5,10.5; L35 13.5,10.5; L36 14.5,10.5; L37 15.5,10.5; L38 16.5,10.5; L39 17.5,10.5; L40 18.5,10.5; L41 19.5,10.5; L42 20.5,10.5; M1 -20.5,9.5; M2 -19.5,9.5; M3 -18.5,9.5; M4 -17.5,9.5; M5 -16.5,9.5; M6 -15.5,9.5; M7 -14.5,9.5; M8 -13.5,9.5; M9 -12.5,9.5; M10 -11.5,9.5; M11 -10.5,9.5; M12 -9.5,9.5; M13 -8.5,9.5; M14 -7.5,9.5; M15 -6.5,9.5; M16 -5.5,9.5; M17 -4.5,9.5; M18 -3.5,9.5; M19 -2.5,9.5; M20 -1.5,9.5; M21 -0.5,9.5; M22 0.5,9.5; M23 1.5,9.5; M24 2.5,9.5; M25 3.5,9.5; M26 4.5,9.5; M27 5.5,9.5; M28 6.5,9.5; M29 7.5,9.5; M30 8.5,9.5; M31 9.5,9.5; M32 10.5,9.5; M33 11.5,9.5; M34 12.5,9.5; M35 13.5,9.5; M36 14.5,9.5; M37 15.5,9.5; M38 16.5,9.5; M39 17.5,9.5; M40 18.5,9.5; M41 19.5,9.5; M42 20.5,9.5; N1 -20.5,8.5; N2 -19.5,8.5; N3 -18.5,8.5; N4 -17.5,8.5; N5 -16.5,8.5; N6 -15.5,8.5; N7 -14.5,8.5; N8 -13.5,8.5; N9 -12.5,8.5; N10 -11.5,8.5; N11 -10.5,8.5; N12 -9.5,8.5; N13 -8.5,8.5; N14 -7.5,8.5; N15 -6.5,8.5; N16 -5.5,8.5; N17 -4.5,8.5; N18 -3.5,8.5; N19 -2.5,8.5; N20 -1.5,8.5; N21 -0.5,8.5; N22 0.5,8.5; N23 1.5,8.5; N24 2.5,8.5; N25 3.5,8.5; N26 4.5,8.5; N27 5.5,8.5; N28 6.5,8.5; N29 7.5,8.5; N30 8.5,8.5; N31 9.5,8.5; N32 10.5,8.5; N33 11.5,8.5; N34 12.5,8.5; N35 13.5,8.5; N36 14.5,8.5; N37 15.5,8.5; N38 16.5,8.5; N39 17.5,8.5; N40 18.5,8.5; N41 19.5,8.5; N42 20.5,8.5; P1 -20.5,7.5; P2 -19.5,7.5; P3 -18.5,7.5; P4 -17.5,7.5; P5 -16.5,7.5; P6 -15.5,7.5; P7 -14.5,7.5; P8 -13.5,7.5; P9 -12.5,7.5; P10 -11.5,7.5; P11 -10.5,7.5; P12 -9.5,7.5; P13 -8.5,7.5; P14 -7.5,7.5; P15 -6.5,7.5; P16 -5.5,7.5; P17 -4.5,7.5; P18 -3.5,7.5; P19 -2.5,7.5; P20 -1.5,7.5; P21 -0.5,7.5; P22 0.5,7.5; P23 1.5,7.5; P24 2.5,7.5; P25 3.5,7.5; P26 4.5,7.5; P27 5.5,7.5; P28 6.5,7.5; P29 7.5,7.5; P30 8.5,7.5; P31 9.5,7.5; P32 10.5,7.5; P33 11.5,7.5; P34 12.5,7.5; P35 13.5,7.5; P36 14.5,7.5; P37 15.5,7.5; P38 16.5,7.5; P39 17.5,7.5; P40 18.5,7.5; P41 19.5,7.5; P42 20.5,7.5; R2 -19.5,6.5; R3 -18.5,6.5; R4 -17.5,6.5; R5 -16.5,6.5; R6 -15.5,6.5; R7 -14.5,6.5; R8 -13.5,6.5; R9 -12.5,6.5; R10 -11.5,6.5; R11 -10.5,6.5; R12 -9.5,6.5; R13 -8.5,6.5; R14 -7.5,6.5; R15 -6.5,6.5; R16 -5.5,6.5; R17 -4.5,6.5; R18 -3.5,6.5; R19 -2.5,6.5; R20 -1.5,6.5; R21 -0.5,6.5; R22 0.5,6.5; R23 1.5,6.5; R24 2.5,6.5; R25 3.5,6.5; R26 4.5,6.5; R27 5.5,6.5; R28 6.5,6.5; R29 7.5,6.5; R30 8.5,6.5; R31 9.5,6.5; R32 10.5,6.5; R33 11.5,6.5; R34 12.5,6.5; R35 13.5,6.5; R36 14.5,6.5; R37 15.5,6.5; R38 16.5,6.5; R39 17.5,6.5; R40 18.5,6.5; R41 19.5,6.5; R42 20.5,6.5; T2 -19.5,5.5; T3 -18.5,5.5; T4 -17.5,5.5; T5 -16.5,5.5; T6 -15.5,5.5; T7 -14.5,5.5; T8 -13.5,5.5; T9 -12.5,5.5; T10 -11.5,5.5; T11 -10.5,5.5; T12 -9.5,5.5; T13 -8.5,5.5; T14 -7.5,5.5; T15 -6.5,5.5; T16 -5.5,5.5; T17 -4.5,5.5; T18 -3.5,5.5; T19 -2.5,5.5; T20 -1.5,5.5; T21 -0.5,5.5; T22 0.5,5.5; T23 1.5,5.5; T24 2.5,5.5; T25 3.5,5.5; T26 4.5,5.5; T27 5.5,5.5; T28 6.5,5.5; T29 7.5,5.5; T30 8.5,5.5; T31 9.5,5.5; T32 10.5,5.5; T33 11.5,5.5; T34 12.5,5.5; T35 13.5,5.5; T36 14.5,5.5; T37 15.5,5.5; T38 16.5,5.5; T39 17.5,5.5; T40 18.5,5.5; T41 19.5,5.5; T42 20.5,5.5; U1 -20.5,4.5; U2 -19.5,4.5; U3 -18.5,4.5; U4 -17.5,4.5; U5 -16.5,4.5; U6 -15.5,4.5; U7 -14.5,4.5; U8 -13.5,4.5; U9 -12.5,4.5; U10 -11.5,4.5; U11 -10.5,4.5; U12 -9.5,4.5; U13 -8.5,4.5; U14 -7.5,4.5; U15 -6.5,4.5; U16 -5.5,4.5; U17 -4.5,4.5; U18 -3.5,4.5; U19 -2.5,4.5; U20 -1.5,4.5; U21 -0.5,4.5; U22 0.5,4.5; U23 1.5,4.5; U24 2.5,4.5; U25 3.5,4.5; U26 4.5,4.5; U27 5.5,4.5; U28 6.5,4.5; U29 7.5,4.5; U30 8.5,4.5; U31 9.5,4.5; U32 10.5,4.5; U33 11.5,4.5; U34 12.5,4.5; U35 13.5,4.5; U36 14.5,4.5; U37 15.5,4.5; U38 16.5,4.5; U39 17.5,4.5; U40 18.5,4.5; U41 19.5,4.5; U42 20.5,4.5; V1 -20.5,3.5; V2 -19.5,3.5; V3 -18.5,3.5; V4 -17.5,3.5; V5 -16.5,3.5; V6 -15.5,3.5; V7 -14.5,3.5; V8 -13.5,3.5; V9 -12.5,3.5; V10 -11.5,3.5; V11 -10.5,3.5; V12 -9.5,3.5; V13 -8.5,3.5; V14 -7.5,3.5; V15 -6.5,3.5; V16 -5.5,3.5; V17 -4.5,3.5; V18 -3.5,3.5; V19 -2.5,3.5; V20 -1.5,3.5; V21 -0.5,3.5; V22 0.5,3.5; V23 1.5,3.5; V24 2.5,3.5; V25 3.5,3.5; V26 4.5,3.5; V27 5.5,3.5; V28 6.5,3.5; V29 7.5,3.5; V30 8.5,3.5; V31 9.5,3.5; V32 10.5,3.5; V33 11.5,3.5; V34 12.5,3.5; V35 13.5,3.5; V36 14.5,3.5; V37 15.5,3.5; V38 16.5,3.5; V39 17.5,3.5; V40 18.5,3.5; V41 19.5,3.5; V42 20.5,3.5; W1 -20.5,2.5; W2 -19.5,2.5; W3 -18.5,2.5; W4 -17.5,2.5; W5 -16.5,2.5; W6 -15.5,2.5; W7 -14.5,2.5; W8 -13.5,2.5; W9 -12.5,2.5; W10 -11.5,2.5; W11 -10.5,2.5; W12 -9.5,2.5; W13 -8.5,2.5; W14 -7.5,2.5; W15 -6.5,2.5; W16 -5.5,2.5; W17 -4.5,2.5; W18 -3.5,2.5; W19 -2.5,2.5; W20 -1.5,2.5; W21 -0.5,2.5; W22 0.5,2.5; W23 1.5,2.5; W24 2.5,2.5; W25 3.5,2.5; W26 4.5,2.5; W27 5.5,2.5; W28 6.5,2.5; W29 7.5,2.5; W30 8.5,2.5; W31 9.5,2.5; W32 10.5,2.5; W33 11.5,2.5; W34 12.5,2.5; W35 13.5,2.5; W36 14.5,2.5; W37 15.5,2.5; W38 16.5,2.5; W39 17.5,2.5; W40 18.5,2.5; W41 19.5,2.5; W42 20.5,2.5; Y1 -20.5,1.5; Y2 -19.5,1.5; Y3 -18.5,1.5; Y4 -17.5,1.5; Y5 -16.5,1.5; Y6 -15.5,1.5; Y7 -14.5,1.5; Y8 -13.5,1.5; Y9 -12.5,1.5; Y10 -11.5,1.5; Y11 -10.5,1.5; Y12 -9.5,1.5; Y13 -8.5,1.5; Y14 -7.5,1.5; Y15 -6.5,1.5; Y16 -5.5,1.5; Y17 -4.5,1.5; Y18 -3.5,1.5; Y19 -2.5,1.5; Y20 -1.5,1.5; Y21 -0.5,1.5; Y22 0.5,1.5; Y23 1.5,1.5; Y24 2.5,1.5; Y25 3.5,1.5; Y26 4.5,1.5; Y27 5.5,1.5; Y28 6.5,1.5; Y29 7.5,1.5; Y30 8.5,1.5; Y31 9.5,1.5; Y32 10.5,1.5; Y33 11.5,1.5; Y34 12.5,1.5; Y35 13.5,1.5; Y36 14.5,1.5; Y37 15.5,1.5; Y38 16.5,1.5; Y39 17.5,1.5; Y40 18.5,1.5; Y41 19.5,1.5; Y42 20.5,1.5
SOT23-DBV = smd 0.55 x 1.2: 1 -0.95,-1.3; 2 0,-1.3; 3 0.95,-1.3; 4 0.95,1.3; 5 -0.95,1.3
SO8 = smd 0.6 x 2.2: 1 -1.905,-2.6; 2 -0.635,-2.6; 3 0.635,-2.6; 4 1.905,-2.6; 5 1.905,2.6; 6 0.635,2.6; 7 -0.635,2.6; 8 -1.905,2.6
L3216C = smd 1.2 x 1.6: 1 -1.5,0; 2 1.5,0
R0402 = smd 0.7 x 0.9: 1 -0.65,0; 2 0.65,0
QFP-7X7-48 = smd 0.3 x 1.2: 1 -2.75,-4.1; 2 -2.25,-4.1; 3 -1.75,-4.1; 4 -1.25,-4.1; 5 -0.75,-4.1; 6 -0.25,-4.1; 7 0.25,-4.1; 8 0.75,-4.1; 9 1.25,-4.1; 10 1.75,-4.1; 11 2.25,-4.1; 12 2.75,-4.1; 25 2.75,4.1; 26 2.25,4.1; 27 1.75,4.1; 28 1.25,4.1; 29 0.75,4.1; 30 0.25,4.1; 31 -0.25,4.1; 32 -0.75,4.1; 33 -1.25,4.1; 34 -1.75,4.1; 35 -2.25,4.1; 36 -2.75,4.1 | smd 1.2 x 0.3: 13 4.1,-2.75; 14 4.1,-2.25; 15 4.1,-1.75; 16 4.1,-1.25; 17 4.1,-0.75; 18 4.1,-0.25; 19 4.1,0.25; 20 4.1,0.75; 21 4.1,1.25; 22 4.1,1.75; 23 4.1,2.25; 24 4.1,2.75; 37 -4.1,2.75; 38 -4.1,2.25; 39 -4.1,1.75; 40 -4.1,1.25; 41 -4.1,0.75; 42 -4.1,0.25; 43 -4.1,-0.25; 44 -4.1,-0.75; 45 -4.1,-1.25; 46 -4.1,-1.75; 47 -4.1,-2.25; 48 -4.1,-2.75 | smd 2 x 2: EXP 0,0
SO-08 = smd 0.6 x 2.2: 1 -1.905,-2.6; 2 -0.635,-2.6; 3 0.635,-2.6; 4 1.905,-2.6; 5 1.905,2.6; 6 0.635,2.6; 7 -0.635,2.6; 8 -1.905,2.6
DCV10_DC/DC = drill 0.8 long: P$1 -3.81,8.89; P$2 -3.81,6.35; P$5 -3.81,-1.27; P$6 -3.81,-3.81; P$7 -3.81,-6.35; P$8 3.81,-6.35; P$14 3.81,8.89
TSSOP16 = smd 0.35 x 1.2: 1 -2.275,-2.925; 2 -1.625,-2.925; 3 -0.975,-2.925; 4 -0.325,-2.925; 5 0.325,-2.925; 6 0.975,-2.925; 7 1.625,-2.925; 8 2.275,-2.925; 9 2.275,2.925; 10 1.625,2.925; 11 0.975,2.925; 12 0.325,2.925; 13 -0.325,2.925; 14 -0.975,2.925; 15 -1.625,2.925; 16 -2.275,2.925; 17 2.895,-2.925; 18 3.545,-2.925; 19 3.545,2.925; 20 2.895,2.925
QFN16 = smd 0.85 x 0.3: 1 -1.475,0.75; 2 -1.475,0.25; 3 -1.475,-0.25; 4 -1.475,-0.75; 9 1.475,-0.75; 10 1.475,-0.25; 11 1.475,0.25; 12 1.475,0.75 | smd 0.3 x 0.85: 5 -0.75,-1.475; 6 -0.25,-1.475; 7 0.25,-1.475; 8 0.75,-1.475; 13 0.75,1.475; 14 0.25,1.475; 15 -0.25,1.475; 16 -0.75,1.475 | smd 1.7 x 1.7: TH 0,0
PAK100/2500-10 = drill 1 pad 1.422: 1 -5.08,-1.27; 2 -5.08,1.27; 3 -2.54,-1.27; 4 -2.54,1.27; 5 0,-1.27; 6 0,1.27; 7 2.54,-1.27; 8 2.54,1.27; 9 5.08,-1.27; 10 5.08,1.27

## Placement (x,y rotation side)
C1  220pF 1%  [C0402]  3.81,85.09 0 top
C2  220pF 1%  [C0402]  3.81,12.7 0 top
C2.  10uF 10%  [SMC_A]  74.93,92.71 180 top
C2.1  10uF 10%  [SMC_A]  74.93,20.32 180 top
C2.2  10uF 10%  [SMC_A]  74.93,68.58 180 top
C2.3  10uF 10%  [SMC_A]  74.93,44.45 180 top
C3  68pF 1%  [C0402]  3.81,77.47 0 top
C4  10nF 10%  [C0402]  73.66,83.82 0 top
C5  10uF 10%  [SMC_A]  20.32,74.93 0 top
C6  100nF 10%  [C0402]  60.96,81.28 0 top
C7  68pF 1%  [C0402]  31.75,96.52 180 top
C8  100nF 10%  [C0402]  52.07,91.44 0 top
C9  68pF 1%  [C0402]  15.24,81.28 0 top
C10  68pF 1%  [C0402]  31.75,90.17 180 top
C11  2.7nF 1%  [C0402]  25.4,85.09 0 top
C12  2.7nF 1%  [C0402]  25.4,80.01 0 top
C13  100nF 10%  [C0402]  60.96,83.82 180 top
C14  100nF 10%  [C0402]  60.96,88.9 0 top
C15  68pF 1%  [C0402]  20.32,80.01 0 top
C16  10uF 10%  [SMC_A]  20.32,77.47 180 top
C17  10nF 10%  [C0402]  78.74,82.55 0 top
C18  10uF 10%  [SMC_A]  44.45,76.2 0 top
C19  10nF 10%  [C0402]  78.74,85.09 0 top
C20  10uF 10%  [SMC_A]  50.8,76.2 180 top
C21  100nF 10%  [C0402]  55.88,86.36 0 top
C22  100nF 10%  [C0402]  55.88,81.28 0 top
C23  100nF 10%  [C0402]  55.88,83.82 0 top
C24  47pF 10%  [C0402]  55.88,78.74 0 top
C25  10uF 10%  [SMC_A]  74.93,96.52 0 top
C26  10nF 10%  [C0402]  73.66,81.28 0 top
C27  10uF 10%  [SMC_A]  48.26,93.98 180 top
C28  100nF 10%  [C0402]  48.26,91.44 0 top
C29  100nF 10%  [C0402]  39.37,91.44 180 top
C30  10uF 10%  [SMC_A]  39.37,96.52 0 top
C31  10nF 10%  [C0402]  48.26,96.52 180 top
C32  100nF 10%  [C0402]  38.1,87.63 180 top
C33  100nF 10%  [C0402]  73.66,86.36 0 top
C34  100nF 10%  [C0402]  78.74,88.9 0 top
C35  100nF 10%  [C0402]  109.22,93.98 180 top
C36  100nF 10%  [C0402]  109.22,91.44 180 top
C37  2,2uF 10%  [SMC_A]  104.14,97.79 180 top
C38  2,2uF 10%  [SMC_A]  104.14,93.98 180 top
C39  10nF 10%  [C0402]  116.84,97.79 0 top
C40  100nF 10%  [C0402]  109.22,97.79 180 top
C41  100nF 10%  [C0402]  115.57,77.47 0 top
C42  100nF 10%  [C0402]  116.84,92.71 180 top
C43  NL 1%  [C0402]  31.75,92.71 180 top
C44  68pF 1%  [C0402]  3.81,5.08 0 top
C45  68pF 1%  [C0402]  15.24,8.89 0 top
C46  68pF 1%  [C0402]  31.75,17.78 180 top
C47  2.7nF 1%  [C0402]  25.4,12.7 0 top
C48  2.7nF 1%  [C0402]  25.4,7.62 0 top
C49  NL 1%  [C0402]  31.75,20.32 180 top
C50  68pF 1%  [C0402]  20.32,7.62 0 top
C51  68pF 1%  [C0402]  31.75,24.13 180 top
C52  10uF 10%  [SMC_A]  20.32,5.08 180 top
C53  10uF 10%  [SMC_A]  20.32,2.54 0 top
C54  10nF 10%  [C0402]  78.74,10.16 0 top
C55  10nF 10%  [C0402]  78.74,12.7 0 top
C56  10nF 10%  [C0402]  48.26,24.13 180 top
C57  10nF 10%  [C0402]  73.66,8.89 0 top
C58  10nF 10%  [C0402]  73.66,11.43 0 top
C59  10uF 10%  [SMC_A]  74.93,24.13 0 top
C60  100nF 10%  [C0402]  60.96,8.89 0 top
C61  100nF 10%  [C0402]  60.96,11.43 180 top
C62  10uF 10%  [SMC_A]  50.8,3.81 180 top
C63  100nF 10%  [C0402]  55.88,13.97 0 top
C64  10uF 10%  [SMC_A]  44.45,3.81 0 top
C65  100nF 10%  [C0402]  55.88,8.89 0 top
C66  100nF 10%  [C0402]  55.88,11.43 0 top
C67  10uF 10%  [SMC_A]  48.26,21.59 180 top
C68  100nF 10%  [C0402]  48.26,19.05 0 top
C69  10uF 10%  [SMC_A]  39.37,24.13 0 top
C70  100nF 10%  [C0402]  39.37,19.05 180 top
C71  100nF 10%  [C0402]  60.96,16.51 0 top
C72  100nF 10%  [C0402]  52.07,19.05 0 top
C73  100nF 10%  [C0402]  38.1,15.24 180 top
C74  47pF 10%  [C0402]  55.88,6.35 0 top
C75  100nF 10%  [C0402]  109.22,19.05 180 top
C76  100nF 10%  [C0402]  109.22,21.59 180 top
C77  100nF 10%  [C0402]  78.74,16.51 0 top
C78  100nF 10%  [C0402]  73.66,13.97 0 top
C79  100nF 10%  [C0402]  116.84,20.32 180 top
C80  100nF 10%  [C0402]  115.57,5.08 0 top
C81  100nF 10%  [C0402]  109.22,25.4 180 top
C82  10nF 10%  [C0402]  116.84,25.4 0 top
C83  2,2uF 10%  [SMC_A]  104.14,25.4 180 top
C84  2,2uF 10%  [SMC_A]  104.14,21.59 180 top
C85  220pF 1%  [C0402]  3.81,60.96 0 top
C86  68pF 1%  [C0402]  3.81,53.34 0 top
C87  68pF 1%  [C0402]  15.24,57.15 0 top
C88  68pF 1%  [C0402]  31.75,66.04 180 top
C89  2.7nF 1%  [C0402]  25.4,60.96 0 top
C90  2.7nF 1%  [C0402]  25.4,55.88 0 top
C91  NL 1%  [C0402]  31.75,68.58 180 top
C92  68pF 1%  [C0402]  20.32,55.88 0 top
C93  68pF 1%  [C0402]  31.75,72.39 180 top
C94  10uF 10%  [SMC_A]  20.32,53.34 180 top
C95  10uF 10%  [SMC_A]  20.32,50.8 0 top
C96  10nF 10%  [C0402]  78.74,58.42 0 top
C97  10nF 10%  [C0402]  78.74,60.96 0 top
C98  10nF 10%  [C0402]  48.26,72.39 180 top
C99  10nF 10%  [C0402]  73.66,57.15 0 top
C100  10nF 10%  [C0402]  73.66,59.69 0 top
C101  10uF 10%  [SMC_A]  74.93,72.39 0 top
C102  100nF 10%  [C0402]  60.96,57.15 0 top
C103  100nF 10%  [C0402]  60.96,59.69 180 top
C104  10uF 10%  [SMC_A]  50.8,52.07 180 top
C105  100nF 10%  [C0402]  55.88,62.23 0 top
C106  10uF 10%  [SMC_A]  44.45,52.07 0 top
C107  100nF 10%  [C0402]  55.88,57.15 0 top
C108  100nF 10%  [C0402]  55.88,59.69 0 top
C109  10uF 10%  [SMC_A]  48.26,69.85 180 top
C110  100nF 10%  [C0402]  48.26,67.31 0 top
C111  10uF 10%  [SMC_A]  39.37,72.39 0 top
C112  100nF 10%  [C0402]  39.37,67.31 180 top
C113  100nF 10%  [C0402]  60.96,64.77 0 top
C114  100nF 10%  [C0402]  52.07,67.31 0 top
C115  100nF 10%  [C0402]  38.1,63.5 180 top
C116  47pF 10%  [C0402]  55.88,54.61 0 top
C117  100nF 10%  [C0402]  109.22,67.31 180 top
C118  100nF 10%  [C0402]  109.22,69.85 180 top
C119  100nF 10%  [C0402]  78.74,64.77 0 top
C120  100nF 10%  [C0402]  73.66,62.23 0 top
C121  100nF 10%  [C0402]  116.84,68.58 180 top
C122  100nF 10%  [C0402]  115.57,53.34 0 top
C123  100nF 10%  [C0402]  109.22,73.66 180 top
C124  10nF 10%  [C0402]  116.84,73.66 0 top
C125  2,2uF 10%  [SMC_A]  104.14,73.66 180 top
C126  2,2uF 10%  [SMC_A]  104.14,69.85 180 top
C127  220pF 1%  [C0402]  3.81,36.83 0 top
C128  68pF 1%  [C0402]  3.81,29.21 0 top
C129  68pF 1%  [C0402]  15.24,33.02 0 top
C130  68pF 1%  [C0402]  31.75,41.91 180 top
C131  2.7nF 1%  [C0402]  25.4,36.83 0 top
C132  2.7nF 1%  [C0402]  25.4,31.75 0 top
C133  NL 1%  [C0402]  31.75,44.45 180 top
C134  68pF 1%  [C0402]  20.32,31.75 0 top
C135  68pF 1%  [C0402]  31.75,48.26 180 top
C136  10uF 10%  [SMC_A]  20.32,29.21 180 top
C137  10uF 10%  [SMC_A]  20.32,26.67 0 top
C138  10nF 10%  [C0402]  78.74,34.29 0 top
C139  10nF 10%  [C0402]  78.74,36.83 0 top
C140  10nF 10%  [C0402]  48.26,48.26 180 top
C141  10nF 10%  [C0402]  73.66,33.02 0 top
C142  10nF 10%  [C0402]  73.66,35.56 0 top
C143  10uF 10%  [SMC_A]  74.93,48.26 0 top
C144  100nF 10%  [C0402]  60.96,33.02 0 top
C145  100nF 10%  [C0402]  60.96,35.56 180 top
C146  10uF 10%  [SMC_A]  50.8,27.94 180 top
C147  100nF 10%  [C0402]  55.88,38.1 0 top
C148  10uF 10%  [SMC_A]  44.45,27.94 0 top
C149  100nF 10%  [C0402]  55.88,33.02 0 top
C150  100nF 10%  [C0402]  55.88,35.56 0 top
C151  10uF 10%  [SMC_A]  48.26,45.72 180 top
C152  100nF 10%  [C0402]  48.26,43.18 0 top
C153  10uF 10%  [SMC_A]  39.37,48.26 0 top
C154  100nF 10%  [C0402]  39.37,43.18 180 top
C155  100nF 10%  [C0402]  60.96,40.64 0 top
C156  100nF 10%  [C0402]  52.07,43.18 0 top
C157  100nF 10%  [C0402]  38.1,39.37 180 top
C158  47pF 10%  [C0402]  55.88,30.48 0 top
C159  100nF 10%  [C0402]  109.22,43.18 180 top
C160  100nF 10%  [C0402]  109.22,45.72 180 top
C161  100nF 10%  [C0402]  78.74,40.64 0 top
C162  100nF 10%  [C0402]  73.66,38.1 0 top
C163  100nF 10%  [C0402]  116.84,44.45 180 top
C164  100nF 10%  [C0402]  115.57,29.21 0 top
C165  100nF 10%  [C0402]  109.22,49.53 180 top
C166  10nF 10%  [C0402]  116.84,49.53 0 top
C167  2,2uF 10%  [SMC_A]  104.14,49.53 180 top
C168  2,2uF 10%  [SMC_A]  104.14,45.72 180 top
E$1  [1297-25]  217.17,49.53 90 top
E$2  [FF1738]  181.61,48.26 0 top
IC1  TPS77001  [SOT23-DBV]  67.31,86.36 90 top
IC2  AD822R  [SO8]  58.42,93.98 0 top
IC3  TPS77001  [SOT23-DBV]  67.31,13.97 90 top
IC4  AD822R  [SO8]  58.42,21.59 0 top
IC5  TPS77001  [SOT23-DBV]  67.31,62.23 90 top
IC6  AD822R  [SO8]  58.42,69.85 0 top
IC7  TPS77001  [SOT23-DBV]  67.31,38.1 90 top
IC8  AD822R  [SO8]  58.42,45.72 0 top
L1  470uH 1%  [L3216C]  3.81,81.28 0 top
L2  470uH 1%  [L3216C]  10.16,81.28 0 top
L3  470uH 1%  [L3216C]  3.81,8.89 0 top
L4  470uH 1%  [L3216C]  10.16,8.89 0 top
L5  470uH 1%  [L3216C]  3.81,57.15 0 top
L6  470uH 1%  [L3216C]  10.16,57.15 0 top
L7  470uH 1%  [L3216C]  3.81,33.02 0 top
L8  470uH 1%  [L3216C]  10.16,33.02 0 top
R1  termination  [R0402]  12.7,85.09 0 top
R2  56k 1%  [R0402]  3.81,88.9 0 top
R3  56k 1%  [R0402]  8.89,85.09 0 top
R4  59k 1%  [R0402]  73.66,88.9 0 top
R5  40k 1%  [R0402]  60.96,86.36 0 top
R6  1k1 1%  [R0402]  3.81,74.93 0 top
R7  1k1 1%  [R0402]  10.16,77.47 180 top
R8  3k57 1%  [R0402]  10.16,74.93 180 top
R9  3k57 1%  [R0402]  15.24,74.93 0 top
R10  10k 1%  [R0402]  57.15,88.9 180 top
R11  3k57 1%  [R0402]  15.24,77.47 180 top
R12  3k57 1%  [R0402]  25.4,82.55 180 top
R13  10k 1%  [R0402]  60.96,76.2 180 top
R14  15 1%  [R0402]  16.51,85.09 180 top
R15  15 1%  [R0402]  31.75,86.36 180 top
R16  6k34 1%  [R0402]  55.88,76.2 0 top
R17  33 5%  [R0402]  78.74,78.74 0 top
R17.  0ohm (non montare)  [R0402]  73.66,77.47 0 top
R17.1  0ohm (non montare)  [R0402]  73.66,5.08 0 top
R17.2  0ohm (non montare)  [R0402]  73.66,53.34 0 top
R17.3  0ohm (non montare)  [R0402]  73.66,29.21 0 top
R18  33 5%  [R0402]  38.1,76.2 180 top
R19  NL  [R0402]  38.1,82.55 180 top
R20  33 5%  [R0402]  25.4,76.2 180 top
R21  33 5%  [R0402]  38.1,78.74 180 top
R22  0ohm (non montare)  [R0402]  78.74,74.93 0 top
R23  33 5%  [R0402]  99.06,83.82 0 top
R24  33 5%  [R0402]  99.06,86.36 0 top
R25  120k 5%  [R0402]  102.87,86.36 180 top
R26  120k 5%  [R0402]  102.87,91.44 180 top
R27  33 5%  [R0402]  115.57,74.93 180 top
R28  0ohm (non montare)  [R0402]  73.66,74.93 180 top
R29  termination  [R0402]  12.7,12.7 0 top
R30  56k 1%  [R0402]  3.81,16.51 0 top
R31  56k 1%  [R0402]  8.89,12.7 0 top
R32  59k 1%  [R0402]  73.66,16.51 0 top
R33  40k 1%  [R0402]  60.96,13.97 0 top
R34  1k1 1%  [R0402]  3.81,2.54 0 top
R35  1k1 1%  [R0402]  10.16,5.08 180 top
R36  3k57 1%  [R0402]  10.16,2.54 180 top
R37  3k57 1%  [R0402]  15.24,2.54 0 top
R38  3k57 1%  [R0402]  15.24,5.08 180 top
R39  3k57 1%  [R0402]  25.4,10.16 180 top
R40  15 1%  [R0402]  16.51,12.7 180 top
R41  15 1%  [R0402]  31.75,13.97 180 top
R42  6k34 1%  [R0402]  55.88,3.81 0 top
R43  10k 1%  [R0402]  60.96,3.81 180 top
R44  10k 1%  [R0402]  57.15,16.51 180 top
R45  33 5%  [R0402]  25.4,3.81 180 top
R46  NL  [R0402]  38.1,10.16 180 top
R47  33 5%  [R0402]  38.1,3.81 180 top
R48  33 5%  [R0402]  38.1,6.35 180 top
R49  33 5%  [R0402]  78.74,6.35 0 top
R50  33 5%  [R0402]  99.06,13.97 0 top
R51  33 5%  [R0402]  99.06,11.43 0 top
R52  33 5%  [R0402]  115.57,2.54 180 top
R53  120k 5%  [R0402]  102.87,19.05 180 top
R54  120k 5%  [R0402]  102.87,13.97 180 top
R55  0ohm (non montare)  [R0402]  73.66,2.54 180 top
R56  0ohm (non montare)  [R0402]  78.74,2.54 0 top
R57  termination  [R0402]  12.7,60.96 0 top
R58  56k 1%  [R0402]  3.81,64.77 0 top
R59  56k 1%  [R0402]  8.89,60.96 0 top
R60  59k 1%  [R0402]  73.66,64.77 0 top
R61  40k 1%  [R0402]  60.96,62.23 0 top
R62  1k1 1%  [R0402]  3.81,50.8 0 top
R63  1k1 1%  [R0402]  10.16,53.34 180 top
R64  3k57 1%  [R0402]  10.16,50.8 180 top
R65  3k57 1%  [R0402]  15.24,50.8 0 top
R66  3k57 1%  [R0402]  15.24,53.34 180 top
R67  3k57 1%  [R0402]  25.4,58.42 180 top
R68  15 1%  [R0402]  16.51,60.96 180 top
R69  15 1%  [R0402]  31.75,62.23 180 top
R70  6k34 1%  [R0402]  55.88,52.07 0 top
R71  10k 1%  [R0402]  60.96,52.07 180 top
R72  10k 1%  [R0402]  57.15,64.77 180 top
R73  33 5%  [R0402]  25.4,52.07 180 top
R74  NL  [R0402]  38.1,58.42 180 top
R75  33 5%  [R0402]  38.1,52.07 180 top
R76  33 5%  [R0402]  38.1,54.61 180 top
R77  33 5%  [R0402]  78.74,54.61 0 top
R78  33 5%  [R0402]  99.06,62.23 0 top
R79  33 5%  [R0402]  99.06,59.69 0 top
R80  33 5%  [R0402]  115.57,50.8 180 top
R81  120k 5%  [R0402]  102.87,67.31 180 top
R82  120k 5%  [R0402]  102.87,62.23 180 top
R83  0ohm (non montare)  [R0402]  73.66,50.8 180 top
R84  0ohm (non montare)  [R0402]  78.74,50.8 0 top
R85  termination  [R0402]  12.7,36.83 0 top
R86  56k 1%  [R0402]  3.81,40.64 0 top
R87  56k 1%  [R0402]  8.89,36.83 0 top
R88  59k 1%  [R0402]  73.66,40.64 0 top
R89  40k 1%  [R0402]  60.96,38.1 0 top
R90  1k1 1%  [R0402]  3.81,26.67 0 top
R91  1k1 1%  [R0402]  10.16,29.21 180 top
R92  3k57 1%  [R0402]  10.16,26.67 180 top
R93  3k57 1%  [R0402]  15.24,26.67 0 top
R94  3k57 1%  [R0402]  15.24,29.21 180 top
R95  3k57 1%  [R0402]  25.4,34.29 180 top
R96  15 1%  [R0402]  16.51,36.83 180 top
R97  15 1%  [R0402]  31.75,38.1 180 top
R98  6k34 1%  [R0402]  55.88,27.94 0 top
R99  10k 1%  [R0402]  60.96,27.94 180 top
R100  10k 1%  [R0402]  57.15,40.64 180 top
R101  33 5%  [R0402]  25.4,27.94 180 top
R102  NL  [R0402]  38.1,34.29 180 top
R103  33 5%  [R0402]  38.1,27.94 180 top
R104  33 5%  [R0402]  38.1,30.48 180 top
R105  33 5%  [R0402]  78.74,30.48 0 top
R106  33 5%  [R0402]  99.06,38.1 0 top
R107  33 5%  [R0402]  99.06,35.56 0 top
R108  33 5%  [R0402]  115.57,26.67 180 top
R109  120k 5%  [R0402]  102.87,43.18 180 top
R110  120k 5%  [R0402]  102.87,38.1 180 top
R111  0ohm (non montare)  [R0402]  73.66,26.67 180 top
R112  0ohm (non montare)  [R0402]  78.74,26.67 0 top
U1  AD7641  [QFP-7X7-48]  46.99,11.43 180 top
U2  SN74LVC2G74  [SO-08]  31.75,6.35 0 top
U3  IL711S-1  [SO-08]  92.71,12.7 270 top
U4  TPS73130DBVT  [SOT23-DBV]  66.04,91.44 90 top
U5  TPS73130DBVT  [SOT23-DBV]  67.31,81.28 90 top
U6  AD7641  [QFP-7X7-48]  46.99,83.82 180 top
U7  TPS73130DBVT  [SOT23-DBV]  67.31,76.2 90 top
U8  TPS73130DBVT  [SOT23-DBV]  66.04,96.52 90 top
U9  SN74LVC2G74  [SO-08]  31.75,78.74 0 top
U10  DCV01_DC/DCDCV010505DP_DC/DC_CONVERTER  [DCV10_DC/DC]  88.9,92.71 270 top
U11  IL711S-1  [SO-08]  92.71,85.09 270 top
U12  IL711S-1  [SO-08]  92.71,77.47 90 top
U13  TPS73130DBVT  [SOT23-DBV]  113.03,96.52 0 top
U14  SN74LVC2G74  [SO-08]  109.22,86.36 90 top
U15  SN65LVDT41PW  [TSSOP16]  107.95,78.74 270 top
U16  IL711S-1  [SO-08]  92.71,5.08 90 top
U17  SN65LVDT41PW  [TSSOP16]  107.95,6.35 270 top
U18  SN74LVC2G74  [SO-08]  109.22,13.97 90 top
U19  TPS73130DBVT  [SOT23-DBV]  113.03,24.13 0 top
U20  TPS73130DBVT  [SOT23-DBV]  66.04,19.05 90 top
U21  TPS73130DBVT  [SOT23-DBV]  67.31,8.89 90 top
U22  TPS73130DBVT  [SOT23-DBV]  66.04,24.13 90 top
U23  TPS73130DBVT  [SOT23-DBV]  67.31,3.81 90 top
U24  DCV01_DC/DCDCV010505DP_DC/DC_CONVERTER  [DCV10_DC/DC]  88.9,20.32 270 top
U25  AD7641  [QFP-7X7-48]  46.99,59.69 180 top
U26  SN74LVC2G74  [SO-08]  31.75,54.61 0 top
U27  IL711S-1  [SO-08]  92.71,60.96 270 top
U28  IL711S-1  [SO-08]  92.71,53.34 90 top
U29  SN65LVDT41PW  [TSSOP16]  107.95,54.61 270 top
U30  SN74LVC2G74  [SO-08]  109.22,62.23 90 top
U31  TPS73130DBVT  [SOT23-DBV]  113.03,72.39 0 top
U32  TPS73130DBVT  [SOT23-DBV]  66.04,67.31 90 top
U33  TPS73130DBVT  [SOT23-DBV]  67.31,57.15 90 top
U34  TPS73130DBVT  [SOT23-DBV]  66.04,72.39 90 top
U35  TPS73130DBVT  [SOT23-DBV]  67.31,52.07 90 top
U36  DCV01_DC/DCDCV010505DP_DC/DC_CONVERTER  [DCV10_DC/DC]  88.9,68.58 270 top
U37  AD7641  [QFP-7X7-48]  46.99,35.56 180 top
U38  SN74LVC2G74  [SO-08]  31.75,30.48 0 top
U39  IL711S-1  [SO-08]  92.71,36.83 270 top
U40  IL711S-1  [SO-08]  92.71,29.21 90 top
U41  SN65LVDT41PW  [TSSOP16]  107.95,30.48 270 top
U42  SN74LVC2G74  [SO-08]  109.22,38.1 90 top
U43  TPS73130DBVT  [SOT23-DBV]  113.03,48.26 0 top
U44  TPS73130DBVT  [SOT23-DBV]  66.04,43.18 90 top
U45  TPS73130DBVT  [SOT23-DBV]  67.31,33.02 90 top
U46  TPS73130DBVT  [SOT23-DBV]  66.04,48.26 90 top
U47  TPS73130DBVT  [SOT23-DBV]  67.31,27.94 90 top
U48  DCV01_DC/DCDCV010505DP_DC/DC_CONVERTER  [DCV10_DC/DC]  88.9,44.45 270 top
U$1  THS4520_QFN16  [QFN16]  20.32,83.82 180 top
U$2  THS4520_QFN16  [QFN16]  20.32,11.43 180 top
U$3  THS4520_QFN16  [QFN16]  20.32,59.69 180 top
U$4  THS4520_QFN16  [QFN16]  20.32,35.56 180 top
X1  2510-  [PAK100/2500-10]  19.05,91.44 0 top
X2  2510-  [PAK100/2500-10]  19.05,67.31 0 top
X3  2510-  [PAK100/2500-10]  19.05,43.18 0 top
X4  2510-  [PAK100/2500-10]  19.05,19.05 0 top
X5  2510-  [PAK100/2500-10]  123.19,85.09 90 top
X6  2510-  [PAK100/2500-10]  19.05,19.05 0 top
X7  2510-  [PAK100/2500-10]  123.19,12.7 90 top
X8  2510-  [PAK100/2500-10]  19.05,67.31 0 top
X9  2510-  [PAK100/2500-10]  123.19,60.96 90 top
X10  2510-  [PAK100/2500-10]  19.05,43.18 0 top
X11  2510-  [PAK100/2500-10]  123.19,36.83 90 top

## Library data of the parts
C1 C2 C2. C2.1-C2.3 C3-C168 L1-L8 R1-R17 R17. R17.1-R17.3 R18-R112 = resistor
E$1 = con-commcon
E$2 = xilinx-virtex-v5
IC1 IC3 IC5 IC7 = texas; MF: TEXAS INSTRUMENTS; MPN: TPS77001DBVT; OC_FARNELL: 8461554; OC_NEWARK: 77C1171
IC2 IC4 IC6 IC8 = analog-devices; MF: ANALOG DEVICES; MPN: AD822BRZ; OC_FARNELL: 1651303
U1 U6 U25 U37 = AD7641
U2 U9 U14 U18 U26 U30 U38 U42 = SN74LVC2G74DCUR_SOP8
U3 U11 U12 U16 U27 U28 U39 U40 = IL711S-1 SOIC8
U4 U5 U7 U8 U13 U19-U23 U31-U35 U43-U47 = TPS73130DBVT
U10 U24 U36 U48 = DCV01_DCDC
U15 U17 U29 U41 = SN65LVDT41PW-TSSOP20
U$1-U$4 = THS4520 QFN16
X1-X11 = con-3m; MF: 3M; MPN: 2510-6002UB; OC_FARNELL: 9838244; OC_NEWARK: 46F4725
